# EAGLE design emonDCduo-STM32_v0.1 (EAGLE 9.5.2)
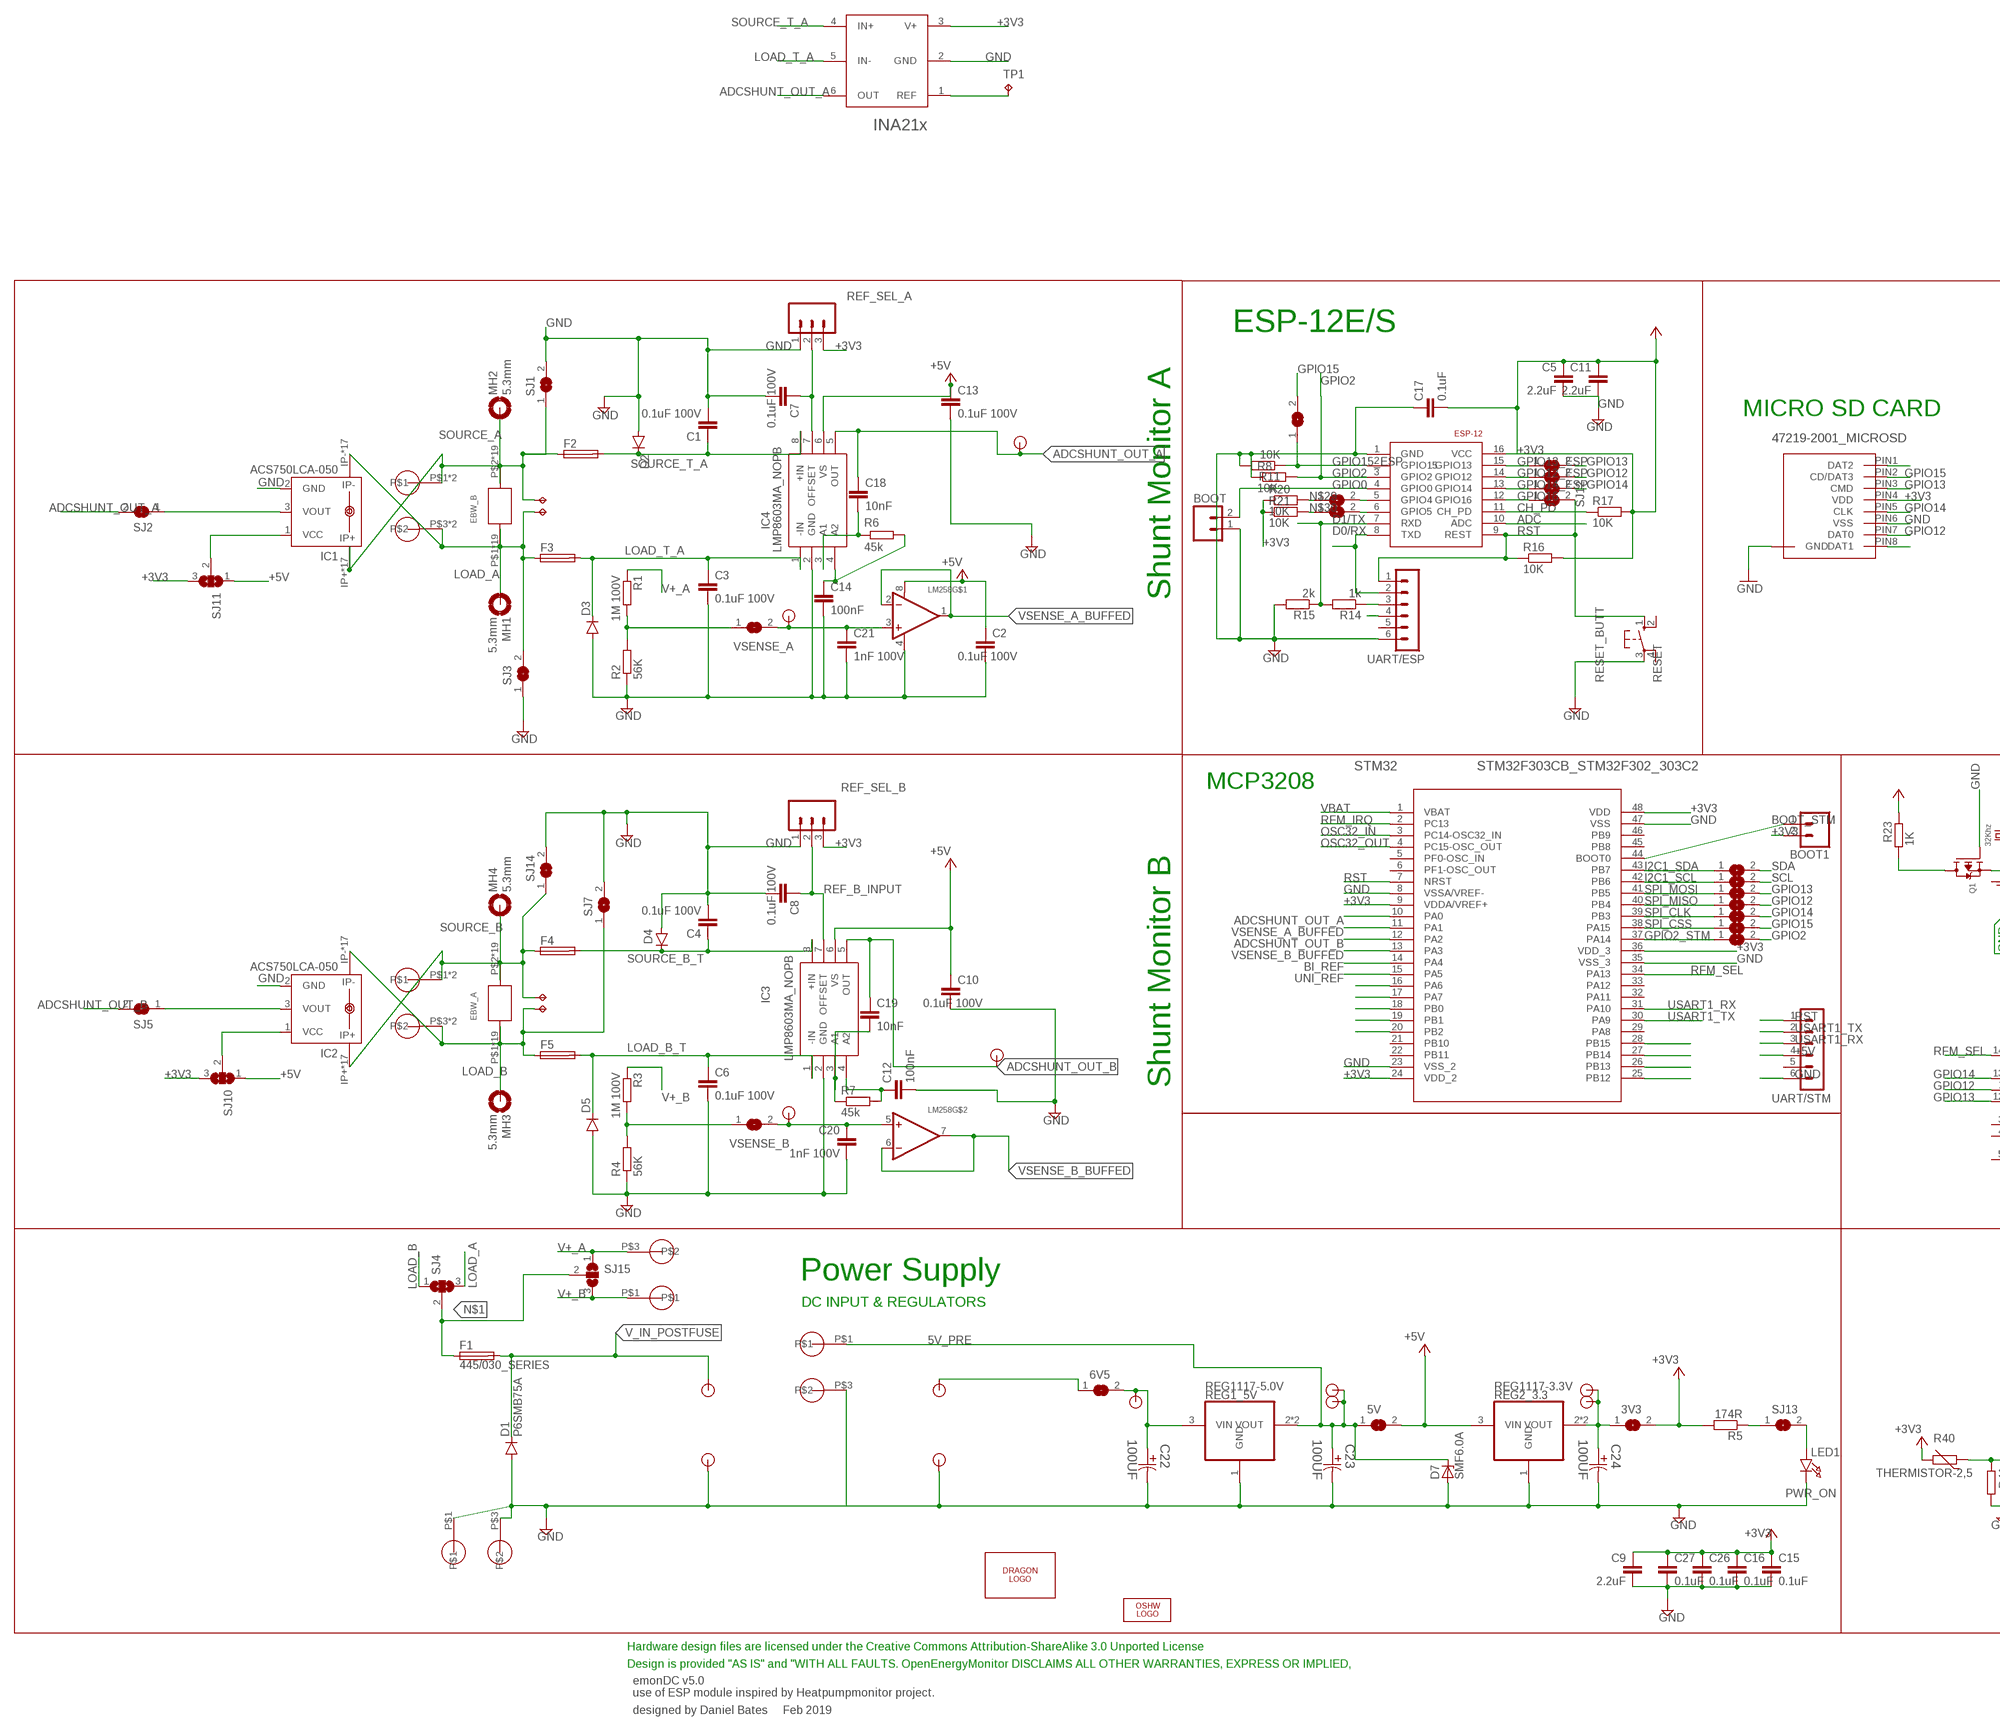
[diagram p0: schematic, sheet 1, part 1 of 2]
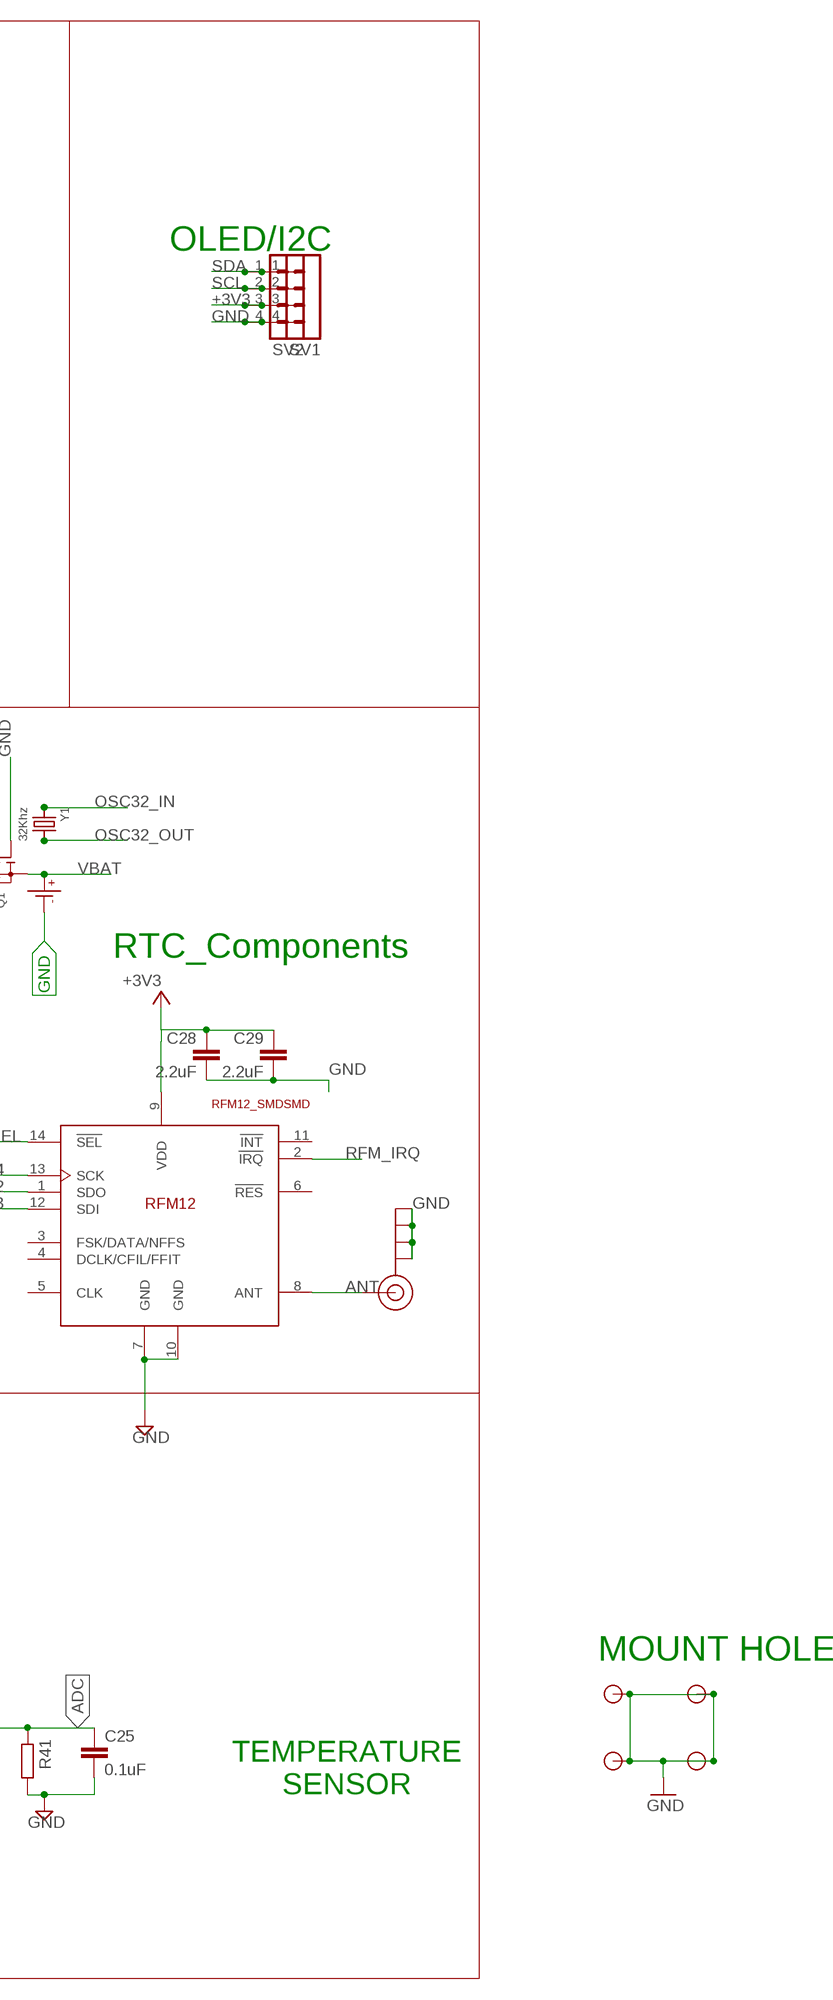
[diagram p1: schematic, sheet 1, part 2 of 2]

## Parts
3V3  SOLDERJUMPERCLOSED  [SOLDERJUMPER_CLOSEDWIRE]
5V  SOLDERJUMPERCLOSED  [SOLDERJUMPER_CLOSEDWIRE]
6V5  SOLDERJUMPERCLOSED  [SOLDERJUMPER_CLOSEDWIRE]
BOOT  M02PTH  [1X02]
BOOT1  M02PTH  [1X02]
C1  0.1uF 100V  C-EUC0603  [C0603]
C2  0.1uF 100V  C-EUC0603  [C0603]
C3  0.1uF 100V  C-EUC0603  [C0603]
C4  0.1uF 100V  C-EUC0603  [C0603]
C5  2.2uF  C-EUC0805  [C0805]
C6  0.1uF 100V  C-EUC0603  [C0603]
C7  0.1uF 100V  C-EUC0603  [C0603]
C8  0.1uF 100V  C-EUC0603  [C0603]
C9  2.2uF  C-EUC0805  [C0805]
C10  0.1uF 100V  C-EUC0603  [C0603]
C11  2.2uF  C-EUC0805  [C0805]
C12  100nF  C-EUC0603  [C0603]
C13  0.1uF 100V  C-EUC0603  [C0603]
C14  100nF  C-EUC0603  [C0603]
C15  0.1uF  C-EUC0603  [C0603]
C16  0.1uF  C-EUC0603  [C0603]
C17  0.1uF  C-EUC0603  [C0603]
C18  10nF  C-EUC0603  [C0603]
C19  10nF  C-EUC0603  [C0603]
C20  1nF 100V  C-EUC0603  [C0603]
C21  1nF 100V  C-EUC0603  [C0603]
C22  100UF  EEE-0JA101WAR-CASE-C  [CAPAE530X610N]
C23  100UF  EEE-0JA101WAR-CASE-C  [CAPAE530X610N]
C24  100UF  EEE-0JA101WAR-CASE-C  [CAPAE530X610N]
C25  0.1uF  C-EUC0603  [C0603]
C26  0.1uF  C-EUC0603  [C0603]
C27  0.1uF  C-EUC0603  [C0603]
C28  2.2uF  C-EUC0805  [C0805]
C29  2.2uF  C-EUC0805  [C0805]
CR1220  CR1220SMD  [CR1220SMD]
D1  P6SMB75A  DIODE-DO214AA  [DO214AA]
D2  P6SMB75A  DIODE-SMB  [SMB]
D3  P6SMB75A  DIODE-SMB  [SMB]
D4  P6SMB75A  DIODE-SMB  [SMB]
D5  P6SMB75A  DIODE-SMB  [SMB]
D7  SMF6.0A  [SOD123F]
EBW_A  EBW_SERIES_15.2MM  [EBW_SERIES_15.2MM]
EBW_B  EBW_SERIES_15.2MM  [EBW_SERIES_15.2MM]
ESP-12  ESP8266_ESP-12  [ESP8266-ESP12]
F1  445/030_SERIES  [445/030_SERIES_LITTELFUSE]
F2  TR5  [TR5]
F3  TR5  [TR5]
F4  TR5  [TR5]
F5  TR5  [TR5]
IC1  ACS750LCA-050  [ACS75050]
IC2  ACS750LCA-050  [ACS75050]
IC3  LMP8603MA_NOPB  [SOIC127P600X175-8N]
IC4  LMP8603MA_NOPB  [SOIC127P600X175-8N]
INA21X_1  INA21X  [SC70]
J$1  SMA_EDGE  [SMA-EDGE]
LED1  PWR_ON  LED1206  [CHIPLED_1206]
LM258  LM358  [SOIC8_150MIL]
LOGO1  OSHW_LOGO_6MILX0200-NT  [OSHW_6X200_NOTEXT]
MH1  5.3mm  MOUNT-PAD-ROUND5.3  [5,3//11-PAD]
MH2  5.3mm  MOUNT-PAD-ROUND5.3  [5,3//11-PAD]
MH3  5.3mm  MOUNT-PAD-ROUND5.3  [5,3//11-PAD]
MH4  5.3mm  MOUNT-PAD-ROUND5.3  [5,3//11-PAD]
MICRO_SD  47219-2001_MICROSD  [47219-2001_MICROSD]
MOUNT_10.16_A  MOLEX_39970-003  [2/10,16]
MOUNT_10.16_B  MOLEX_39970-003  [2/10,16]
Q1  MOSFET-P  [SOT23-R]
R1  1M 100V  R-EU_0207/2V  [0207/2V]
R2  56K  R-EU_0207/2V  [0207/2V]
R3  1M 100V  R-EU_0207/2V  [0207/2V]
R4  56K  R-EU_0207/2V  [0207/2V]
R5  174R  R-EU_R0603  [R0603]
R6  45k  R-EU_R0603  [R0603]
R7  45k  R-EU_R0603  [R0603]
R8  10K  R-EU_R0603  [R0603]
R11  10K  R-EU_R0603  [R0603]
R14  1k  R-EU_R0603  [R0603]
R15  2k  R-EU_R0603  [R0603]
R16  10K  R-EU_R0603  [R0603]
R17  10K  R-EU_R0603  [R0603]
R20  10K  R-EU_R0603  [R0603]
R21  10K  R-EU_R0603  [R0603]
R23  1K  R-EU_R0603  [R0603]
R40  THERMISTOR-2,5  [RS-2,5]
R41  R-EU_0207/2V  [0207/2V]
REF_SEL_A  455-1750-1-ND  CONN_03  [1X03]
REF_SEL_B  455-1750-1-ND  CONN_03  [1X03]
REG1_5V  REG1117-5.0V  REG1117  [SOT223]
REG2_3.3  REG1117-3.3V  REG1117  [SOT223]
RESET  RESET_BUTT  10-XX  [B3F-10XX]
SJ1  SJ  [SJ]
SJ2  SJ  [SJ]
SJ3  SJ  [SJ]
SJ4  SJ2W  [SJ_2]
SJ5  SJ  [SJ]
SJ6  SJTINY  [SJ-SMALL]
SJ7  SJ  [SJ]
SJ8  SOLDERJUMPERCLOSED  [SOLDERJUMPER_CLOSEDWIRE]
SJ9  SOLDERJUMPERCLOSED  [SOLDERJUMPER_CLOSEDWIRE]
SJ10  SJ2W  [SJ_2]
SJ11  SJ2W  [SJ_2]
SJ12  SJTINY  [SJ-SMALL]
SJ13  SOLDERJUMPERCLOSED  [SOLDERJUMPER_CLOSEDWIRE]
SJ14  SJ  [SJ]
SJ15  SJ2W  [SJ_2]
SJ16  SJTINY  [SJ-SMALL]
SJ17  SJTINY  [SJ-SMALL]
SJ18  SJTINY  [SJ-SMALL]
SJ19  SJTINY  [SJ-SMALL]
SJ20  SJTINY  [SJ-SMALL]
SJ21  SJTINY  [SJ-SMALL]
SJ22  SJTINY  [SJ-SMALL]
SJ23  SJTINY  [SJ-SMALL]
SJ24  SJTINY  [SJ-SMALL]
SJ25  SJTINY  [SJ-SMALL]
SJ26  SJTINY  [SJ-SMALL]
SJ27  SJTINY  [SJ-SMALL]
STM32  STM32F303CB_STM32F302_303C2  [STM32F303CB_LQFP48-7X7MM]
SV1  MA04-1  [MA04-1]
SV2  MA04-1  [MA04-1]
TP1  TPPAD1-13  [P1-13]
TP8  TPPAD1-13Y  [P1-13Y]
TP9  TPPAD1-13Y  [P1-13Y]
TP10  TPPAD1-13Y  [P1-13Y]
TP11  TPPAD1-13Y  [P1-13Y]
U$1  TP0.8MM  [TP0.8]
U$2  2212S-02SG-85  TP_2_LONG  [TP0.8_X2]
U$3  2212S-02SG-85  TP_2_LONG  [TP0.8_X2]
U$4  TP0.8MM  [TP0.8]
U$5  TP0.8MM  [TP0.8]
U$6  TP0.8MM  [TP0.8]
U$7  TP0.8MM  [TP0.8]
U$8  TP0.8MM  [TP0.8]
U$9  TP0.8MM  [TP0.8]
U$10  2212S-02SG-85  TP_2_LONG  [TP0.8_X2]
U$11  2212S-02SG-85  TP_2_LONG  [TP0.8_X2]
U$12  5MMBLOCK  [2/5.08]
U$13  5MMBLOCK  [2/5.08]
U$14  RFM12_SMDSMD  [RFM12]
U$18  TP0.8MM  [TP0.8]
U$19  TP0.8MM  [TP0.8]
U$21  5MMBLOCK  [2/5.08]
U$22  TP3.5MM  [TP3.5]
U$23  TP3.5MM  [TP3.5]
U$24  TP3.5MM  [TP3.5]
U$25  TP3.5MM  [TP3.5]
U$26  DRAGON  [DRAGON_LOGO]
UART/ESP  UART/ESP  MA06-1  [MA06-1]
UART/STM  UART/STM  MA06-1  [MA06-1]
Y1  32Khz  CRYSTAL8X3.8SMT  [CRYSTAL_8X3.8]

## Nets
3.3V_PRE [thick_power]: 3V3.1 C24.1 REG2_3.3.2(VOUT) REG2_3.3.4(VOUT) U$8.P$1 U$19.P$1
5V_PRE [thick_power]: 5V.1 C23.1 D7.C REG1_5V.2(VOUT) REG1_5V.4(VOUT) U$7.P$1 U$12.P$1 U$18.P$1
6.5V [thick_power]: 6V5.2 C22.1 REG1_5V.3(VIN) U$9.P$1
+3V3 [thin_power]: 3V3.2 BOOT1.2 C5.1 C9.1 C11.1 C15.1 C16.1 C17.2 C26.1 C27.1 C28.1 C29.1 ESP-12.16(VCC) INA21X_1.3(V+) MICRO_SD.PIN4(VDD) R5.2 R16.2 R17.2 R20.1 R21.1 R23.2 R40.2 REF_SEL_A.3 REF_SEL_B.3 SJ10.3 SJ11.3 STM32.9(VDDA/VREF+) STM32.24(VDD_2) STM32.36(VDD_3) STM32.48(VDD) SV1.3 SV2.3 U$14.9(VDD)
+3V3_BAT [thick_power]: Q1.3(D) R23.1
+5V [thick_power]: 5V.2 C2.1 C10.1 C13.1 IC3.6(VS) IC4.6(VS) LM258.8(V+) REG2_3.3.3(VIN) SJ10.1 SJ11.1 UART/ESP.4 UART/STM.4
ADC: C25.1 ESP-12.10(ADC) R40.1 R41.2
ADCSHUNT_OUT_A: C18.1 IC4.5(OUT) INA21X_1.6(OUT) SJ2.2 STM32.10(PA0) U$6.P$1
ADCSHUNT_OUT_B: C19.1 IC3.5(OUT) SJ5.2 STM32.12(PA2) U$5.P$1
ANT: J$1.SIG(SIGNAL) U$14.8(ANT)
BI_REF: STM32.14(PA4)
BOOT_STM: BOOT1.1 STM32.44(BOOT0)
CH_PD: ESP-12.11(CH_PD) R17.1
D0/RX: ESP-12.8(TXD) UART/ESP.2
D1/TX: ESP-12.7(RXD) R14.2 R15.1
GND: BOOT.1 C1.2 C2.2 C3.2 C4.2 C5.2 C6.2 C7.2 C8.2 C9.2 C10.2 C11.2 C12.2 C13.2 C14.2 C15.2 C16.2 C17.1 C20.2 C21.2 C22.2 C23.2 C24.2 C25.2 C26.2 C27.2 C28.2 C29.2 CR1220.P-(P$-) D1.A D2.A D3.A D4.A D5.A D7.A ESP-12.1(GND) IC1.2(GND) IC2.2(GND) IC3.2(GND) IC4.2(GND) INA21X_1.2(GND) J$1.GND@0(GND) J$1.GND@1(GND) J$1.GND@2(GND) J$1.GND@3(GND) LED1.C LM258.4(V-) MICRO_SD.P$1(GND) MICRO_SD.P$2(GND) MICRO_SD.P$3(GND) MICRO_SD.P$4(GND) MICRO_SD.PIN6(VSS) Q1.1(G) R2.1 R4.1 R8.1 R11.2 R15.2 R41.1 REF_SEL_A.1 REF_SEL_B.1 REG1_5V.1(GND) REG2_3.3.1(GND) RESET.3(P) SJ1.2 SJ3.1 SJ7.2 SJ14.2 STM32.8(VSSA/VREF-) STM32.23(VSS_2) STM32.35(VSS_3) STM32.47(VSS) SV1.4 SV2.4 U$3.P$1 U$3.P$2 U$11.P$1 U$11.P$2 U$12.P$3 U$13.P$1 U$13.P$3 U$14.7(GND) U$14.10(GND) U$22.P$1 U$23.P$1 U$24.P$1 U$25.P$1 UART/ESP.6 UART/STM.6
GPIO0: BOOT.2 ESP-12.4(GPIO0)
GPIO2: ESP-12.3(GPIO2) R8.2 SJ21.2
GPIO2_STM: SJ21.1 STM32.37(PA14)
GPIO12: MICRO_SD.PIN7(DAT0) SJ17.2 SJ26.2 U$14.1(SDO)
GPIO12_ESP: ESP-12.14(GPIO12) SJ26.1
GPIO13: MICRO_SD.PIN3(CMD) SJ18.2 SJ25.2 U$14.12(SDI)
GPIO13_ESP: ESP-12.15(GPIO13) SJ25.1
GPIO14: MICRO_SD.PIN5(CLK) SJ16.2 SJ27.2 U$14.13(SCK)
GPIO14_ESP: ESP-12.13(GPIO14) SJ27.1
GPIO15: MICRO_SD.PIN2(CD/DAT3) SJ6.2 SJ22.2
GPIO15_ESP: ESP-12.2(GPIO15) R11.1 SJ22.1
GPIO16: ESP-12.12(GPIO16) SJ12.1
I2C1_SCL: SJ19.1 STM32.42(PB6)
I2C1_SDA: SJ20.1 STM32.43(PB7)
LOAD_A [HV]: EBW_B.P$1 EBW_B.P$3 EBW_B.P$4 EBW_B.P$5 EBW_B.P$6 EBW_B.P$7 EBW_B.P$8 EBW_B.P$9 EBW_B.P$10 EBW_B.P$11 EBW_B.P$12 EBW_B.P$13 EBW_B.P$14 EBW_B.P$15 EBW_B.P$16 EBW_B.P$17 EBW_B.P$33 EBW_B.P$34 EBW_B.P$35 F3.1 IC1.IP- IC1.IP-@2(IP-) IC1.IP-@3(IP-) IC1.IP-@4(IP-) IC1.IP-@5(IP-) IC1.IP-@6(IP-) IC1.IP-@7(IP-) IC1.IP-@8(IP-) IC1.IP-@9(IP-) IC1.IP-@10(IP-) IC1.IP-@11(IP-) IC1.IP-@12(IP-) IC1.IP-@13(IP-) IC1.IP-@14(IP-) IC1.IP-@15(IP-) IC1.IP-@16(IP-) IC1.IP-@17(IP-) MH1.B5,5(MOUNT) MOUNT_10.16_A.P$3 MOUNT_10.16_A.P$4 SJ3.2 SJ4.3 TP10.TP
LOAD_B [HV]: EBW_A.P$1 EBW_A.P$3 EBW_A.P$4 EBW_A.P$5 EBW_A.P$6 EBW_A.P$7 EBW_A.P$8 EBW_A.P$9 EBW_A.P$10 EBW_A.P$11 EBW_A.P$12 EBW_A.P$13 EBW_A.P$14 EBW_A.P$15 EBW_A.P$16 EBW_A.P$17 EBW_A.P$33 EBW_A.P$34 EBW_A.P$35 F5.1 IC2.IP- IC2.IP-@2(IP-) IC2.IP-@3(IP-) IC2.IP-@4(IP-) IC2.IP-@5(IP-) IC2.IP-@6(IP-) IC2.IP-@7(IP-) IC2.IP-@8(IP-) IC2.IP-@9(IP-) IC2.IP-@10(IP-) IC2.IP-@11(IP-) IC2.IP-@12(IP-) IC2.IP-@13(IP-) IC2.IP-@14(IP-) IC2.IP-@15(IP-) IC2.IP-@16(IP-) IC2.IP-@17(IP-) MH3.B5,5(MOUNT) MOUNT_10.16_B.P$3 MOUNT_10.16_B.P$4 SJ4.1 SJ7.1 TP8.TP
LOAD_B_T [thin_power]: C6.1 D5.C F5.2 IC3.1(-IN)
LOAD_T_A [thin_power]: C3.1 D3.C F3.2 IC4.1(-IN) INA21X_1.5(IN-)
N$1: F1.P$1 F1.P$2 SJ4.2 SJ15.2
N$3: C14.1 IC4.4(A2) R6.2
N$4: C18.2 IC4.3(A1) R6.1
N$5: R5.1 SJ13.1
N$6: LED1.A SJ13.2
N$7: MICRO_SD.PIN1(DAT2)
N$9: STM32.18(PB0)
N$10: STM32.19(PB1)
N$11: STM32.20(PB2)
N$15: STM32.25(PB12)
N$17: STM32.26(PB13)
N$20: STM32.27(PB14)
N$22: STM32.28(PB15)
N$23: STM32.17(PA7)
N$24: STM32.16(PA6)
N$25: C19.2 IC3.3(A1) R7.1
N$27: C12.1 IC3.4(A2) R7.2
N$29: R20.2 SJ23.1
N$30: R21.2 SJ24.1
N$32: MICRO_SD.PIN8(DAT1)
N$36: R14.1 UART/ESP.3
N$37: INA21X_1.1(REF) TP1.TP
OSC32_IN: STM32.3(PC14-OSC32_IN) Y1.P$1
OSC32_OUT: STM32.4(PC15-OSC_OUT) Y1.P$4
REF_A_INPUT: C7.1 IC4.7(OFFSET) REF_SEL_A.2
REF_B_INPUT: C8.1 IC3.7(OFFSET) REF_SEL_B.2
RFM_IRQ: STM32.2(PC13) U$14.2(!IRQ)
RFM_SEL: STM32.34(PA13) U$14.14(!SEL)
RST: ESP-12.9(REST) R16.1 RESET.1(S) SJ12.2 STM32.7(NRST) UART/ESP.1 UART/STM.1
SCL: ESP-12.6(GPIO5) SJ19.2 SJ24.2 SV1.2 SV2.2
SDA: ESP-12.5(GPIO4) SJ20.2 SJ23.2 SV1.1 SV2.1
SOURCE_A [HV]: EBW_B.P$2 EBW_B.P$18 EBW_B.P$19 EBW_B.P$20 EBW_B.P$21 EBW_B.P$22 EBW_B.P$23 EBW_B.P$24 EBW_B.P$25 EBW_B.P$26 EBW_B.P$27 EBW_B.P$28 EBW_B.P$29 EBW_B.P$30 EBW_B.P$31 EBW_B.P$32 EBW_B.P$36 EBW_B.P$37 EBW_B.P$38 F2.1 IC1.IP+ IC1.IP+@2(IP+) IC1.IP+@3(IP+) IC1.IP+@4(IP+) IC1.IP+@5(IP+) IC1.IP+@6(IP+) IC1.IP+@7(IP+) IC1.IP+@8(IP+) IC1.IP+@9(IP+) IC1.IP+@10(IP+) IC1.IP+@11(IP+) IC1.IP+@12(IP+) IC1.IP+@13(IP+) IC1.IP+@14(IP+) IC1.IP+@15(IP+) IC1.IP+@16(IP+) IC1.IP+@17(IP+) MH2.B5,5(MOUNT) MOUNT_10.16_A.P$1 MOUNT_10.16_A.P$2 SJ1.1 TP11.TP
SOURCE_B [HV]: EBW_A.P$2 EBW_A.P$18 EBW_A.P$19 EBW_A.P$20 EBW_A.P$21 EBW_A.P$22 EBW_A.P$23 EBW_A.P$24 EBW_A.P$25 EBW_A.P$26 EBW_A.P$27 EBW_A.P$28 EBW_A.P$29 EBW_A.P$30 EBW_A.P$31 EBW_A.P$32 EBW_A.P$36 EBW_A.P$37 EBW_A.P$38 F4.1 IC2.IP+ IC2.IP+@2(IP+) IC2.IP+@3(IP+) IC2.IP+@4(IP+) IC2.IP+@5(IP+) IC2.IP+@6(IP+) IC2.IP+@7(IP+) IC2.IP+@8(IP+) IC2.IP+@9(IP+) IC2.IP+@10(IP+) IC2.IP+@11(IP+) IC2.IP+@12(IP+) IC2.IP+@13(IP+) IC2.IP+@14(IP+) IC2.IP+@15(IP+) IC2.IP+@16(IP+) IC2.IP+@17(IP+) MH4.B5,5(MOUNT) MOUNT_10.16_B.P$1 MOUNT_10.16_B.P$2 SJ14.1 TP9.TP
SOURCE_B_T [thin_power]: C4.1 D4.C F4.2 IC3.8(+IN)
SOURCE_T_A [thin_power]: C1.1 D2.C F2.2 IC4.8(+IN) INA21X_1.4(IN+)
SPI_CLK: SJ16.1 STM32.39(PB3)
SPI_CSS: SJ6.1 STM32.38(PA15)
SPI_MISO: SJ17.1 STM32.40(PB4)
SPI_MOSI: SJ18.1 STM32.41(PB5)
UNI_REF: STM32.15(PA5)
USART1_RX: STM32.31(PA10) UART/STM.3
USART1_TX: STM32.30(PA9) UART/STM.2
V+_A [HV]: R1.1 SJ15.1 U$21.P$3
V+_B [HV]: R3.1 SJ15.3 U$21.P$1
V_IN_POSTFUSE [HV]: D1.C F1.P$3 F1.P$4 U$2.P$1 U$2.P$2
VBAT: CR1220.P+(P$+) Q1.2(S) STM32.1(VBAT)
VCC_ACS_A: IC1.1(VCC) SJ11.2
VCC_ACS_B: IC2.1(VCC) SJ10.2
VOUT_ACS_A: IC1.3(VOUT) SJ2.1
VOUT_ACS_B: IC2.3(VOUT) SJ5.1
VOUT_POST_SWITCHING: 6V5.1 U$10.P$1 U$10.P$2
VSENSE_A: R1.2 R2.2 SJ8.1
VSENSE_A_BUFFED: LM258.1(OUT) LM258.2(-IN) STM32.11(PA1)
VSENSE_A_TP: C21.1 LM258.3(+IN) SJ8.2 U$1.P$1
VSENSE_B: R3.2 R4.2 SJ9.1
VSENSE_B_BUFFED: LM258.6(-IN) LM258.7(OUT) STM32.13(PA3)
VSENSE_B_TP: C20.1 LM258.5(+IN) SJ9.2 U$4.P$1
Unconnected: RESET.2(S1) RESET.4(P1) STM32.5(PF0-OSC_IN) STM32.6(PF1-OSC_OUT) STM32.21(PB10) STM32.22(PB11) STM32.29(PA8) STM32.32(PA11) STM32.33(PA12) STM32.45(PB8) STM32.46(PB9) U$14.3(FSK/DATA/NFFS) U$14.4(DCLK/CFIL/FFIT) U$14.5(CLK) U$14.6(!RES) U$14.11(!INT) UART/ESP.5 UART/STM.5

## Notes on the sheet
- ESP-12E/S
- MICRO SD CARD
- OLED/I2C
- Shunt Monitor A
- MCP3208
- RTC_Components
- Shunt Monitor B
- Power Supply
- DC INPUT & REGULATORS
- MOUNT HOLES
- TEMPERATURE
  SENSOR
- Hardware design files are licensed under the Creative Commons Attribution-ShareAlike 3.0 Unported License
- Design is provided "AS IS" and "WITH ALL FAULTS. OpenEnergyMonitor DISCLAIMS ALL OTHER WARRANTIES, EXPRESS OR IMPLIED,
- emonDC v5.0
  use of ESP module inspired by Heatpumpmonitor project.
- designed by Daniel Bates     Feb 2019

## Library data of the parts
3V3 5V 6V5 SJ8 SJ9 SJ13 = microbuilder:SOLDERJUMPER: SMD Solder JUMPER
BOOT BOOT1 = SparkFun:M02: Header 2
C1-C4 C6-C8 C10 C13 C14 C18-C21 = rcl:C-EU: CAPACITOR, European symbol; MPN: C1608X7S2A104K080AB; SPICEPREFIX: C
C5 C9 C11 C12 C15-C17 C25-C29 = rcl:C-EU: CAPACITOR, European symbol; SPICEPREFIX: C
C22-C24 = Panasonic-EEE0_EEE1_EEE2_EEEFC:EEE-: Aluminum Electrolytic Capacitors,Surface Mount Type; MPN: EEE-0JA101WAR; OC_FARNELL: 2284723; OC_NEWARK: 53W3731; PACKAGE: CASE-C; SUPPLIER: PANASONIC; TOLERANCE: 20%; VOLTAGERATING: 6.3V
CR1220 = IotaWatt_parts:CR1220SMD: CR1220 Battery SMD; MPN: Harwin S8411-45R
D1-D5 = diode:DIODE-: DIODE
D7 = smf_10:SMF*A: SMF Series TVS Diodes; MF: Littelfuse; MPN: SMF6.0A; OC_FARNELL: unknown; OC_NEWARK: unknown
EBW_A EBW_B = EBW series SHUNT:EBW_SERIES_15.2MM
ESP-12 = ESP8266-ESP12:ESP8266_ESP-12
F1 = LITTELFUSE 455:030 SERIES:445/030_SERIES: MPN 04450001N
F2-F5 = fuse_db:TR5: FUSE; MF: LITTELFUSE; MPN: 56000001009; OC_FARNELL: 1185363; OC_NEWARK: unknown
IC1 IC2 = allegro:ACS750*CA-050: Current Sensor display layer 49 Reference in BRD and place VIAs on circles Source: www.allegromicro.com/datafile/0750-050.pdf; MF: ALLEGRO MICROSYSTEMS, INC.; MPN: ACS750LCA-050; OC_FARNELL: 1457176; OC_NEWARK: 61H4464
IC3 IC4 = LMP8603MA_NOPB:LMP8603MA_NOPB: 60-V, Bi-Directional, Low- or High-Side, Voltage Output Current Sensing Amplifier Source: Datasheet; DESCRIPTION: 60-V, Bi-Directional, Low- or High-Side, Voltage Output Current Sensing Amplifier; HEIGHT: 1.75mm; MANUFACTURER_NAME: Texas Instruments; MANUFACTURER_PART_NUMBER: LMP8603MA/NOPB; RS_PART_NUMBER: 7616334P; RS_PRICE-STOCK: http://uk.rs-online.com/web/p/products/7616334P
INA21X_1 = ina21x:INA21X: Texas Instruments INA21x
J$1 = SparkFun-Connectors:SMA_EDGE: SMA Antenna Connector End launch SMA connector. The paste layer has been removed so that the connector can be hand soldered onto the board after reflow.
LED1 = microbuilder:LED: LED
LM258 = microbuilder:LM358: LM358 Dual Operational Amplifier Digikey: LM358AMXFSCT-ND
LOGO1 = ohw-logo:OSHW_LOGO_6MIL; OC_FARNELL: unknown
MH1-MH4 = holes-db:MOUNT-PAD-ROUND: MOUNTING PAD, round
MICRO_SD = MOLEX 47219-2001:47219-2001_MICROSD
MOUNT_10.16_A MOUNT_10.16_B = 10.16mm terminal block:MOLEX_39970-003
Q1 = microbuilder:MOSFET-P: P-Channel Mosfet LEGEND VDS: Voltage Drain-Source ID: Drain Current RDS(ON): Drain-Source On-State Resistance VGS(TH): Gate-Source Threshold Voltage CISS: Drain-Source Input Capacitance SOT-23 Name VDS ID RDS(ON) VGS(TH) CISS Order Number IRLML5103 30V 760mA 600 mOhm -- 75pF @ 25V Digikey: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
R1 R3 = rcl7:R-EU_: RESISTOR, European symbol; MPN: MCMF006FF1004A50
R2 R4 = rcl7:R-EU_: RESISTOR, European symbol; MPN: MCMF006FF7502A50
R5 = rcl:R-EU_: RESISTOR, European symbol; SPICEPREFIX: R
R6-R8 R11 R14-R17 R20 R21 = rcl:R-EU_: RESISTOR, European symbol
R23 = rcl@1:R-EU_: RESISTOR, European symbol
R40 = varistor:THERMISTOR: THERMISTOR
R41 = rcl7:R-EU_: RESISTOR, European symbol
REF_SEL_A REF_SEL_B = SparkFun-Connectors:CONN_03: Multi connection point. Often used as Generic Header-pin footprint for 0.1 inch spaced/style header connections On any of the 0.1 inch spaced packages, you can populate with these: Break Away Headers - Straight (PRT-00116) Break Away Male Headers - Right Angle (PRT-00553) Female Headers (PRT-00115)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; MF: MULTICOMP; MPN: 2212S-02SG-85; OC_FARNELL: 1593458; PROD_ID: XXX-00000
REG1_5V = burr-brown-db:REG1117: 800mA and 1A Low Dropout (LDO) Positive Regulator 1.8V, 2.5V, 2.85V, 3.3V, 5V, and Adj; MF: TEXAS INSTRUMENTS; MPN: REG1117-5.0; OC_FARNELL: 1097566; OC_NEWARK: 14P6981
REG2_3.3 = burr-brown-db:REG1117: 800mA and 1A Low Dropout (LDO) Positive Regulator 1.8V, 2.5V, 2.85V, 3.3V, 5V, and Adj; MF: TEXAS INSTRUMENTS; MPN: REG1117-3.3; OC_FARNELL: 1097566; OC_NEWARK: 14P6981
RESET = switch-omron:10-XX: OMRON SWITCH; MPN: FSM4JH; OC_FARNELL: 155598
SJ1-SJ3 SJ5 SJ7 SJ14 = jumper:SJ: SMD solder JUMPER
SJ4 SJ10 SJ11 SJ15 = jumper:SJ2W: SMD solder JUMPER
SJ6 SJ12 SJ16-SJ27 = jumper-con_db:SJ: SMD solder JUMPER
STM32 = stm32hw05:STM32F303CB_STM32F302_303C2; MANUFACTURER_PART_NUMBER: stm32f302_303c2; VENDOR: STMicroelectronics
SV1 SV2 = con-lstb-db:MA04-1: PIN HEADER; MF: MULTICOMP; MPN: 2212S-04SG-85; OC_FARNELL: 1593460; OC_NEWARK: unknown
TP1 TP8-TP11 = testpad:TP: Test pad
U$1 U$4-U$9 U$18 U$19 U$22-U$25 = testpad_db:TP
U$2 U$3 U$10 U$11 = testpad_db:TP_2_LONG; MPN: 2212S-02SG-85
U$12 U$13 U$21 = 5mm terminal block:5MMBLOCK; MF: LUMBERG; MPN: KRM_02; OC_FARNELL: 1177875
U$14 = rfm12b _ rfm69cw:RFM12_SMD: RFM12 is a low costing ISM band transceiver module implemented with unique PLL. It works signal ranges from 315/433/868/915MHZ bands, comply with FCC, ETSI regulation. The SPI interface is used to communicate with microcontroller for parameter setting.
U$26 = DRAGON_LOGO:DRAGON
UART/ESP UART/STM = JeeLabs:MA06-1: PIN HEADER
Y1 = microbuilder:CRYSTAL: Crystals

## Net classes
0 default: width 0.203 mm, drill 0.5 mm, clearance 0.178 mm
1 power: width 0.254 mm, drill 0.5 mm, clearance 0.203 mm
2 thin_power: width 0.254 mm, drill 0.5 mm, clearance 0.203 mm
3 thick_power: width 0.406 mm, drill 0.5 mm, clearance 0.203 mm
4 HV: width 0.406 mm, drill 0.5 mm, clearance 0.762 mm

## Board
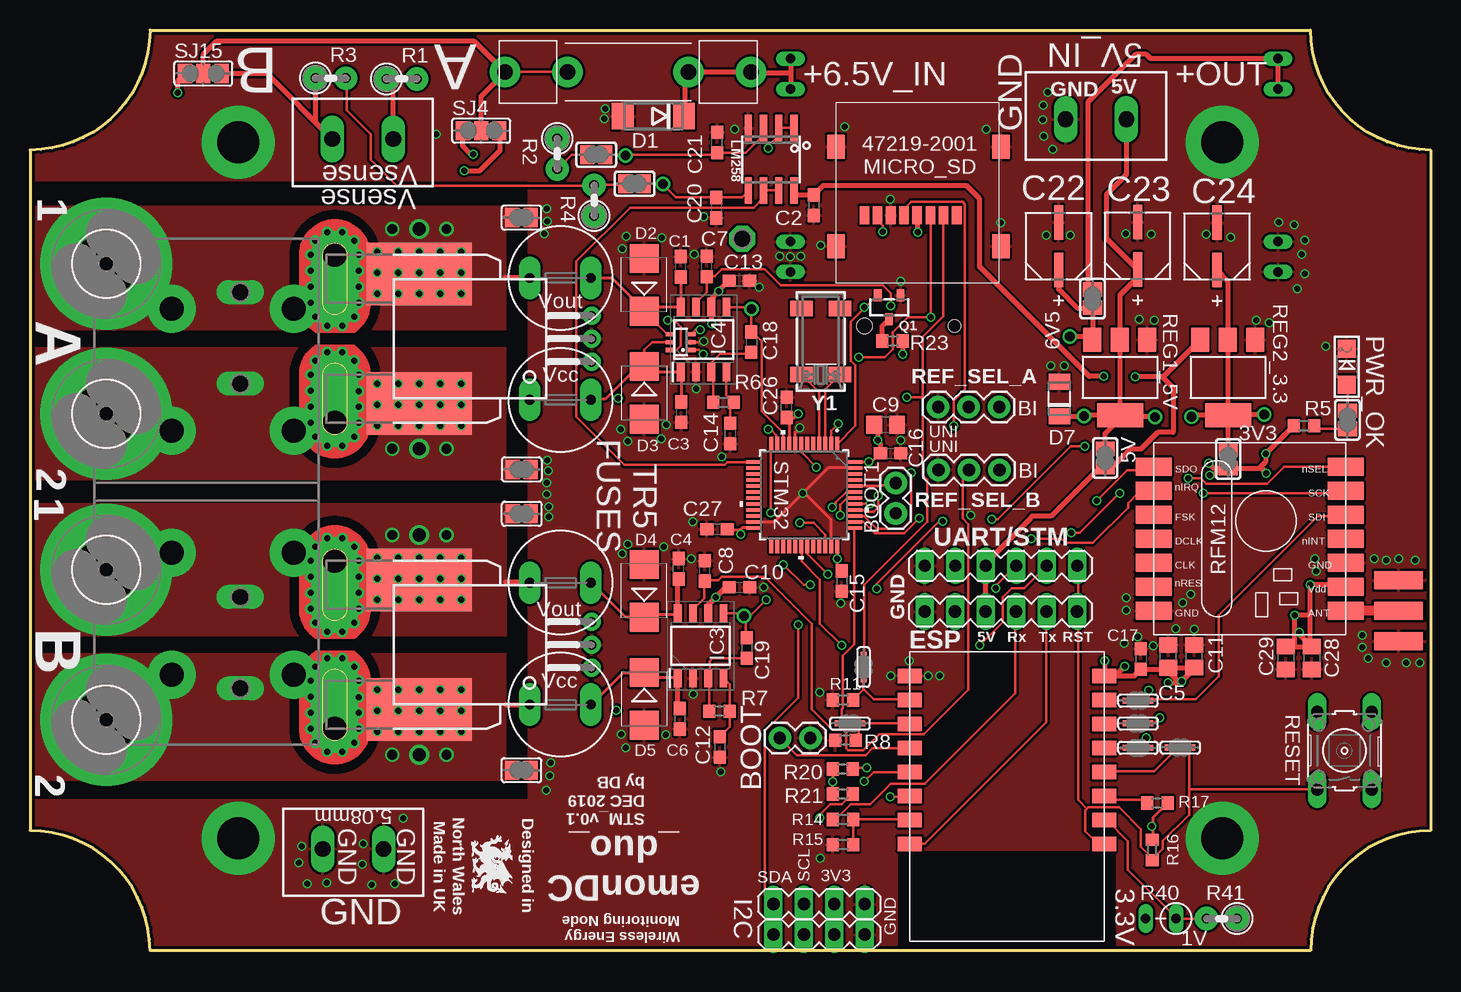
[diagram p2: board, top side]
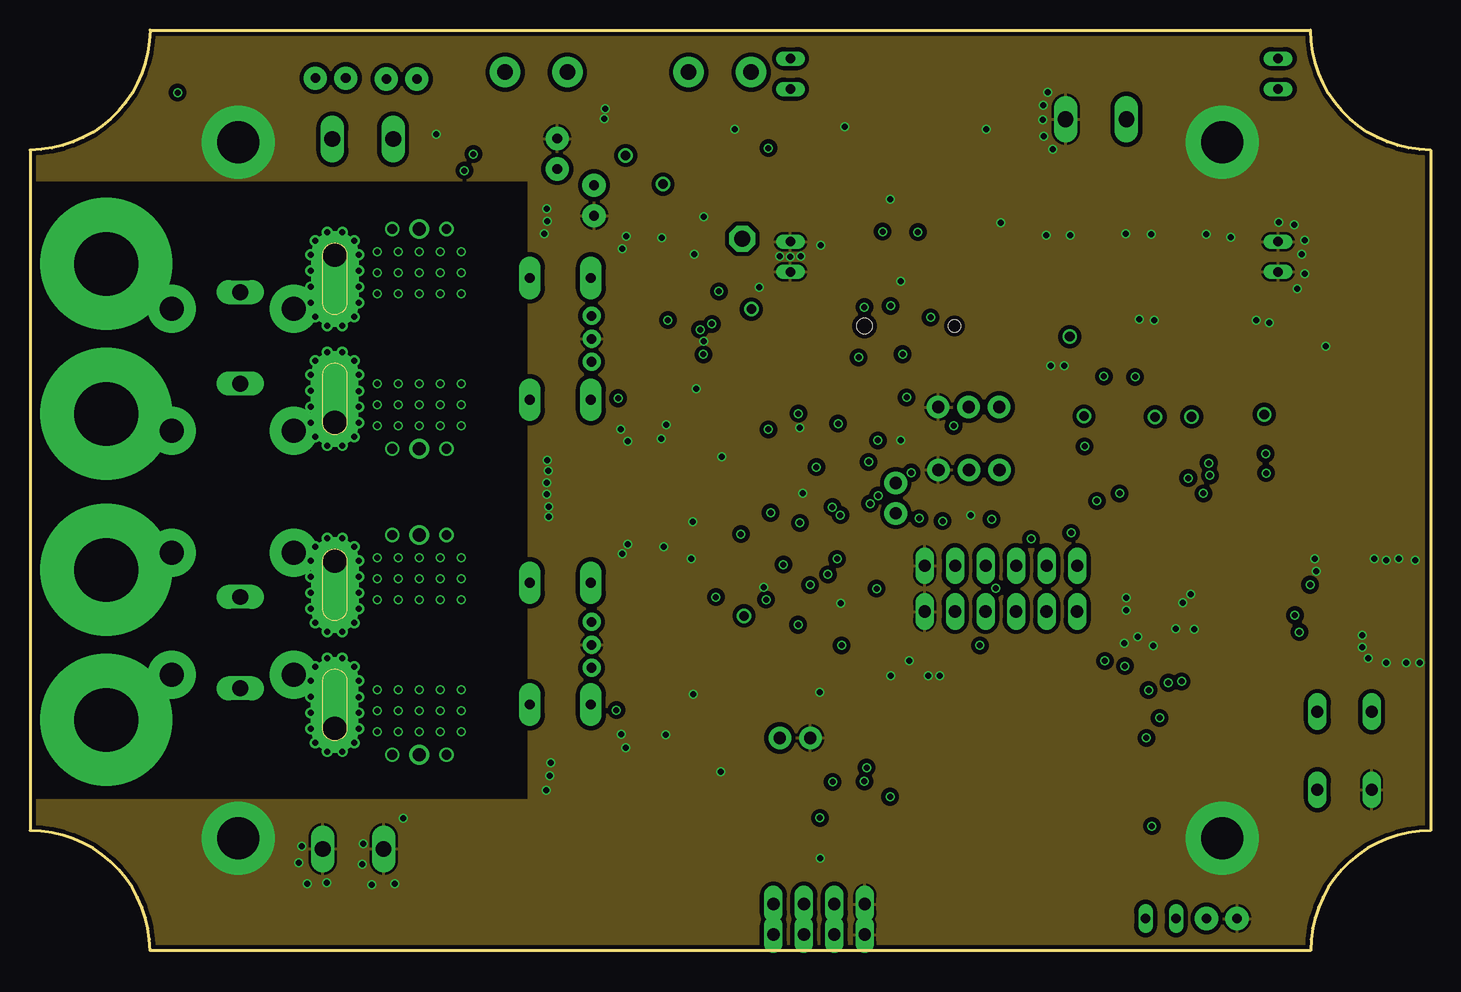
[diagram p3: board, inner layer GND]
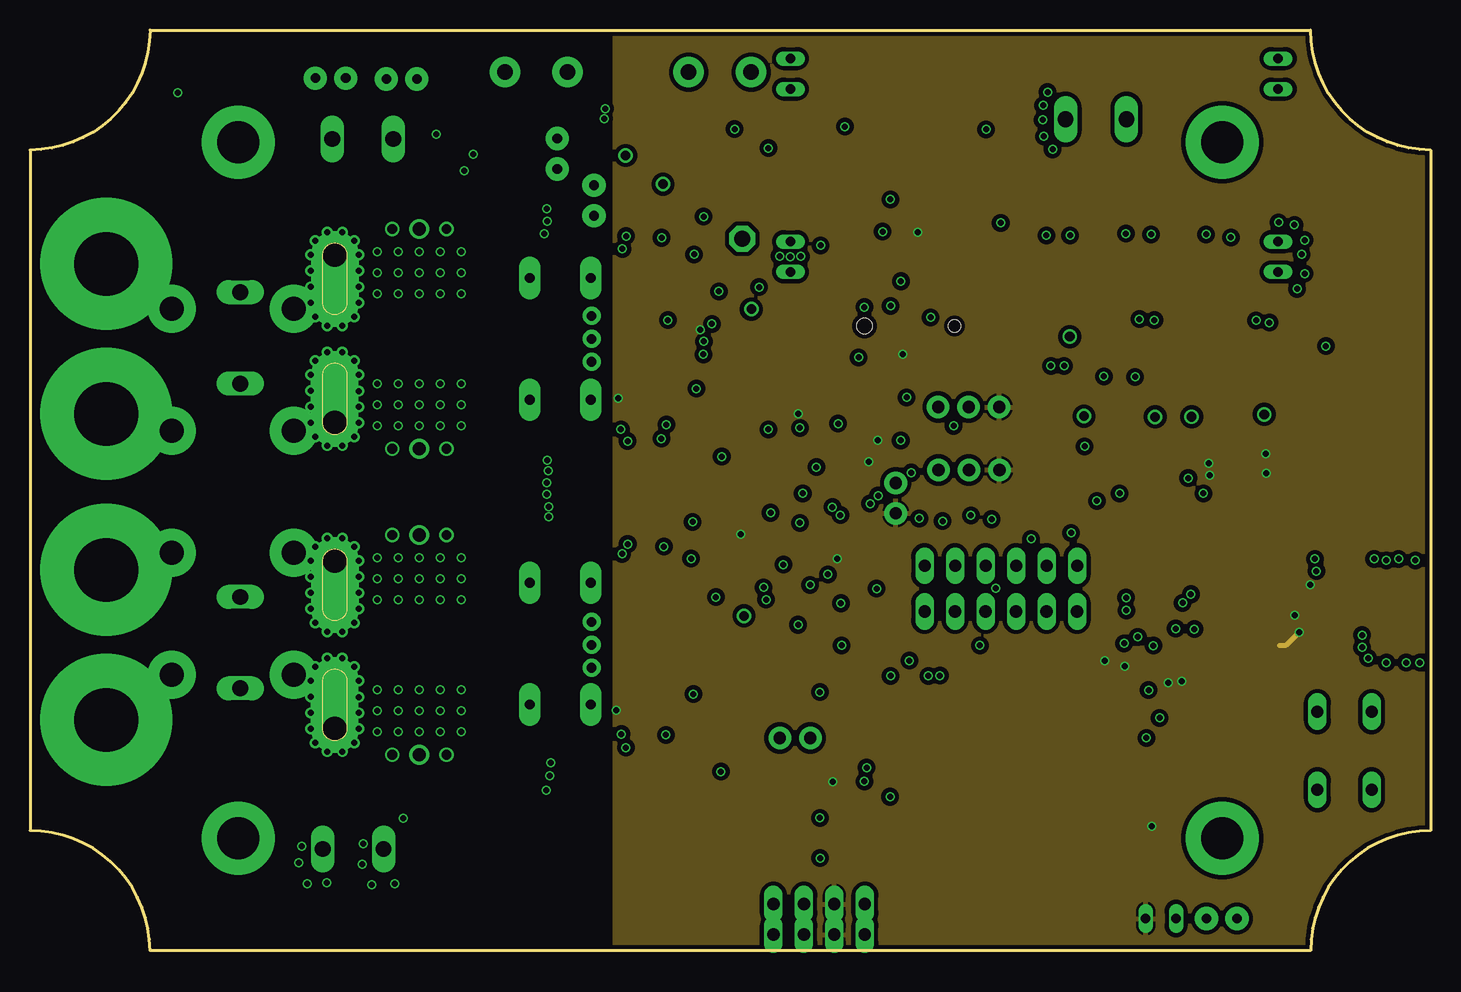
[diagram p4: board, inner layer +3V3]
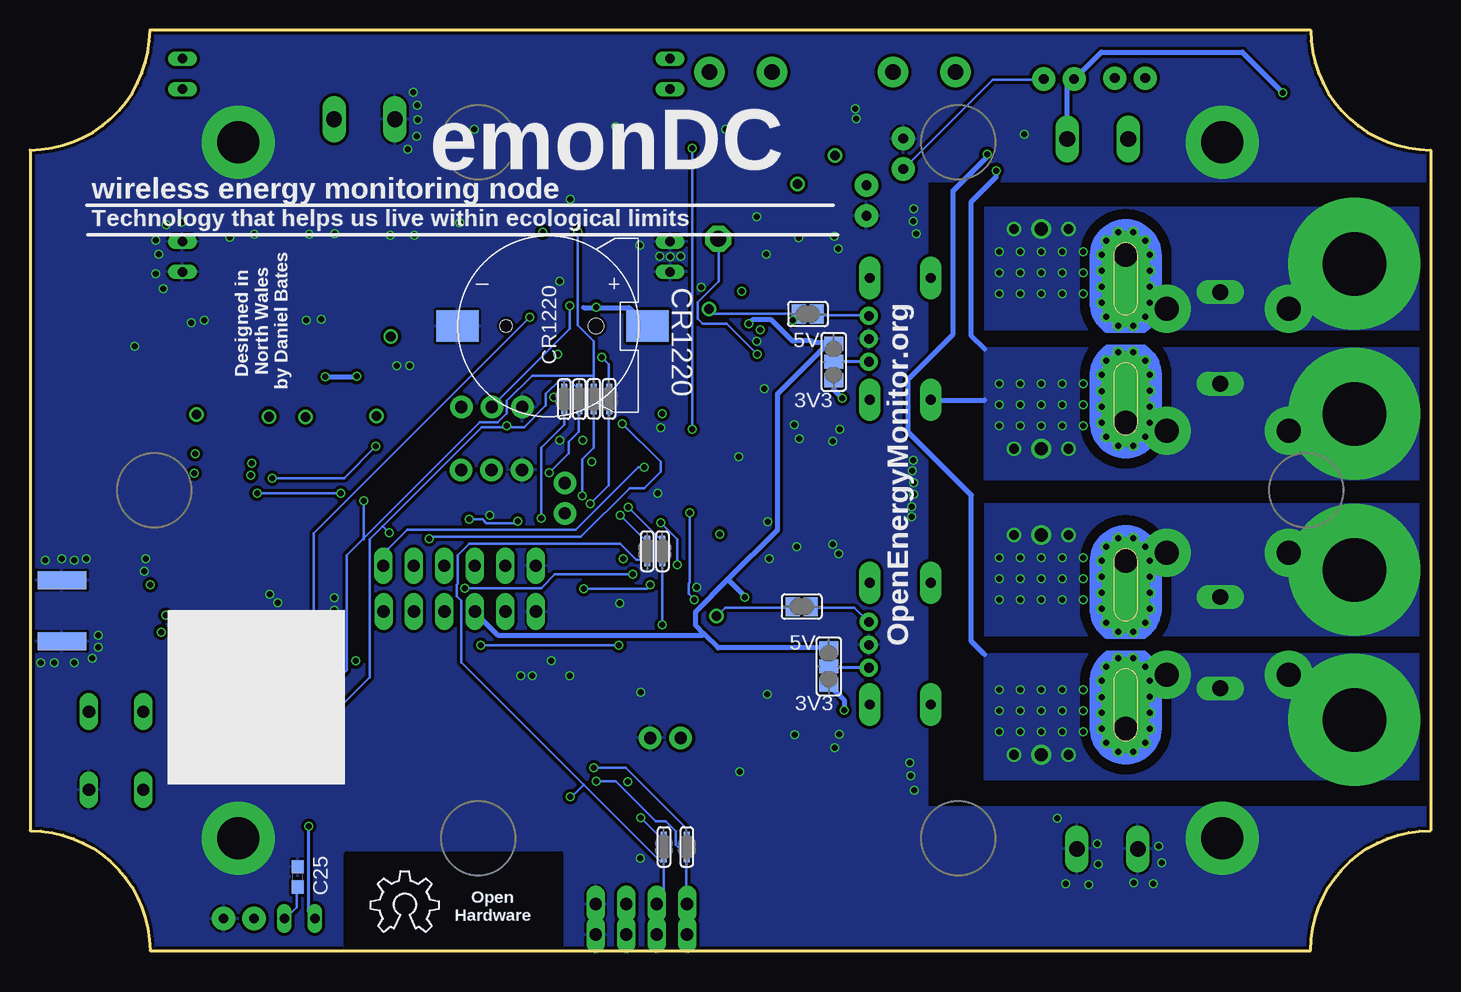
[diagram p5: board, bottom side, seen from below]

Size 116.71 x 76.71 mm. Coordinates in mm from the lower left corner, seen from the top.
Outline: 0,66.71 0,10 arc-90 10,0 106.71,0 arc-90 116.71,10 116.71,66.71 arc-90 106.71,76.71 10,76.71 arc-90 0,66.71
Copper layers (1+2*15+16): Top 0.035mm / dielectric 0.2mm / GND 0.0175mm / dielectric 1.1mm / +3V3 0.0175mm / dielectric 0.2mm / Bottom 0.035mm
Design rules "jlcpcb *": minimum track width 6mil, minimum drill 0.35mm, track to track 7mil, track to pad 7mil, pad to pad 7mil, via to via 0.1mm, smd to smd 2mil, copper to edge 10mil, drill to drill 10mil, minimum pad ring 3mil, minimum via ring 3mil, stop-mask expansion 2mil, vias tented up to drill 25mil, thermal gap 8mil
tRestrict: area 72.5,0.5 to 90.3,8.1
bRestrict: area 72.5,0.4 to 90.3,8

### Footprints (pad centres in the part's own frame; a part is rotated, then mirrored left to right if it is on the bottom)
SOLDERJUMPER_CLOSEDWIRE = smd 1.168 x 1.6: 1 -0.762,0; 2 0.762,0 | smd 0.635 x 0.203: WIRE 0,0
1X02 = drill 1.016 pad 1.88: 1 0,0; 2 2.54,0
C0603 = smd 1.1 x 1: 1 -0.85,0; 2 0.85,0
C0805 = smd 1.3 x 1.5: 1 -0.95,0; 2 0.95,0
CAPAE530X610N = smd 2.87 x 0.762: 1 -1.981,0; 2 1.981,0
CR1220SMD = smd 3.54 x 2.6: P+ 8.3,0; P- -7.55,0 | hole 1: -3.5,0 | hole 1.3: 4,0
DO214AA = smd 1.8 x 2.2: A 2.55,0; C -2.55,0
SMB = smd 2.4 x 2.4: A 2.2,0; C -2.2,0
SOD123F = smd 1.34 x 1.8: A 1.43,0; C -1.43,0
EBW_SERIES_15.2MM = smd 5.2 x 8.75: P$1 -5.4,0; P$2 5.4,0 | drill 0.5: P$3 -3.75,3.5; P$4 -3.75,1.75; P$5 -3.75,0; P$6 -3.75,-1.75; P$7 -3.75,-3.5; P$8 -5.5,3.5; P$9 -5.5,1.75; P$10 -5.5,0; P$11 -5.5,-1.75; P$12 -5.5,-3.5; P$13 -7.25,3.5; P$14 -7.25,1.75; P$15 -7.25,0; P$16 -7.25,-1.75; P$17 -7.25,-3.5; P$18 7.25,1.75; P$19 7.25,3.5; P$20 7.25,0; P$21 7.25,-1.75; P$22 7.25,-3.5; P$23 5.5,3.5; P$24 5.5,1.75; P$25 5.5,0; P$26 5.5,-1.75; P$27 5.5,-3.5; P$28 3.75,3.5; P$29 3.75,1.75; P$30 3.75,0; P$31 3.75,-1.75; P$32 3.75,-3.5 | drill 0.8: P$33 -9.155,2.258; P$35 -9.155,-2.258; P$36 9.155,2.258; P$38 9.155,-2.258 | drill 1.1: P$34 -9.155,0; P$37 9.155,0
ESP8266-ESP12 = smd 2 x 1.2: 1 16.2,2; 2 16.2,4; 3 16.2,6; 4 16.2,8; 5 16.2,10; 6 16.2,12; 7 16.2,14; 8 16.2,16; 9 0,16; 10 0,14; 11 0,12; 12 0,10; 13 0,8; 14 0,6; 15 0,4; 16 0,2
445/030_SERIES_LITTELFUSE = drill 1.3 pad 2.54: P$1 -10.25,0; P$2 -5.05,0; P$3 10.25,0; P$4 5.05,0
TR5 = drill 0.813 pad 1.778 long: 1 -2.54,0; 2 2.54,0
ACS75050 = drill 0.8 pad 1.5: 1 -1.91,-21.4; 2 0,-21.4; 3 1.91,-21.4 | drill 2 pad 4 offset: IP+ 7,0; IP- -7,0 | drill 0.5 pad 0.9: IP+@2 8.89,-0.635; IP+@3 8.89,0.635; IP+@4 8.175,1.625; IP+@5 7,2; IP+@6 5.675,2; IP+@7 4.325,2; IP+@8 3,2; IP+@9 1.825,1.625; IP+@10 1.1,0.625; IP+@11 1.1,-0.625; IP+@12 1.825,-1.625; IP+@13 3,-2; IP+@14 4.325,-2; IP+@15 5.675,-2; IP+@16 7,-2; IP+@17 8.175,-1.625; IP-@2 -8.89,-0.635; IP-@3 -8.89,0.635; IP-@4 -8.175,1.625; IP-@5 -7,2; IP-@6 -5.675,2; IP-@7 -4.325,2; IP-@8 -3,2; IP-@9 -1.825,1.625; IP-@10 -1.1,0.625; IP-@11 -1.1,-0.625; IP-@12 -1.825,-1.625; IP-@13 -3,-2; IP-@14 -4.35,-2; IP-@15 -5.675,-2; IP-@16 -7,-2; IP-@17 -8.175,-1.625
SOIC127P600X175-8N = smd 1.528 x 0.65: 1 -2.711,1.905; 2 -2.711,0.635; 3 -2.711,-0.635; 4 -2.711,-1.905; 5 2.711,-1.905; 6 2.711,-0.635; 7 2.711,0.635; 8 2.711,1.905
SC70 = smd 0.35 x 0.8: 1 -0.65,-0.85; 2 0,-0.85; 3 0.65,-0.85; 4 0.65,0.85; 5 0,0.85; 6 -0.65,0.85
SMA-EDGE = smd 1.524 x 4.064: GND@0 0,0; GND@1 5.08,0; SIG 2.54,0 | smd 1.524 x 4.064 bottom: GND@2 0,0; GND@3 5.08,0
CHIPLED_1206 = smd 1.5 x 1.5: A 0,-1.496; C 0,1.496
SOIC8_150MIL = smd 0.6 x 2.2: 1 -1.905,-2.6; 2 -0.635,-2.6; 3 0.635,-2.6; 4 1.905,-2.6; 5 1.905,2.6; 6 0.635,2.6; 7 -0.635,2.6; 8 -1.905,2.6
5,3//11-PAD = drill 5.3 pad 11: B5,5 0,0
47219-2001_MICROSD = smd 1.45 x 2: P$1 0,0; P$2 13.75,0; P$3 0,8.3; P$4 13.75,8.3 | smd 0.8 x 1.5: PIN1 10.08,2.6; PIN2 8.98,2.6; PIN3 7.88,2.6; PIN4 6.78,2.6; PIN5 5.68,2.6; PIN6 4.58,2.6; PIN7 3.48,2.6; PIN8 2.38,2.6
2/10,16 = drill 2 pad 4: P$1 -5.08,0; P$2 -5.08,10.16; P$3 5.08,0; P$4 5.08,10.16
SOT23-R = smd 0.635 x 1.016: 1 -0.95,-1; 2 0.95,-1; 3 0,1
0207/2V = drill 0.813 pad 1.93: 1 -1.27,0; 2 1.27,0
R0603 = smd 1 x 1.1: 1 -0.85,0; 2 0.85,0
RS-2,5 = drill 0.813 long: 1 -1.27,0; 2 1.27,0
1X03 = drill 1.016 pad 1.88: 1 0,0; 2 2.54,0; 3 5.08,0
SOT223 = smd 1.499 x 2.007: 1 -2.261,-3.15; 2 0.025,-3.15; 3 2.311,-3.15 | smd 3.81 x 2.007: 4 0,3.15
B3F-10XX = drill 1.016 long: 1 -3.251,2.261; 2 3.251,2.261; 3 -3.251,-2.261; 4 3.251,-2.261
SJ = smd 1.168 x 1.6: 1 -0.762,0; 2 0.762,0
SJ_2 = smd 1.168 x 1.6: 1 -1.524,0; 2 0,0; 3 1.524,0
SJ-SMALL = smd 1.016 x 0.508: 1 -0.762,0; 2 0.762,0
STM32F303CB_LQFP48-7X7MM = smd 1.194 x 0.305: 1 -4.25,2.75; 2 -4.25,2.25; 3 -4.25,1.75; 4 -4.25,1.25; 5 -4.25,0.75; 6 -4.25,0.25; 7 -4.25,-0.25; 8 -4.25,-0.75; 9 -4.25,-1.25; 10 -4.25,-1.75; 11 -4.25,-2.25; 12 -4.25,-2.75; 25 4.25,-2.75; 26 4.25,-2.25; 27 4.25,-1.75; 28 4.25,-1.25; 29 4.25,-0.75; 30 4.25,-0.25; 31 4.25,0.25; 32 4.25,0.75; 33 4.25,1.25; 34 4.25,1.75; 35 4.25,2.25; 36 4.25,2.75 | smd 0.305 x 1.194: 13 -2.75,-4.25; 14 -2.25,-4.25; 15 -1.75,-4.25; 16 -1.25,-4.25; 17 -0.75,-4.25; 18 -0.25,-4.25; 19 0.25,-4.25; 20 0.75,-4.25; 21 1.25,-4.25; 22 1.75,-4.25; 23 2.25,-4.25; 24 2.75,-4.25; 37 2.75,4.25; 38 2.25,4.25; 39 1.75,4.25; 40 1.25,4.25; 41 0.75,4.25; 42 0.25,4.25; 43 -0.25,4.25; 44 -0.75,4.25; 45 -1.25,4.25; 46 -1.75,4.25; 47 -2.25,4.25; 48 -2.75,4.25
MA04-1 = drill 1.016 long: 1 -3.81,0; 2 -1.27,0; 3 1.27,0; 4 3.81,0
P1-13 = drill 1.321 pad 2.159 octagon: TP 0,0
P1-13Y = drill 1.321 pad 1.905 long: TP 0,0
TP0.8 = drill 0.8: P$1 0,0
TP0.8_X2 = drill 0.8 long: P$1 0,0; P$2 0,2.54
2/5.08 = drill 1.3 long: P$1 -2.54,0; P$3 2.54,0
RFM12 = smd 1.5 x 3: 1 -5,-10; 2 -3,-10; 3 -1,-10; 4 1,-10; 5 3,-10; 6 5,-10; 7 7,-10; 8 7,6; 9 5,6; 10 3,6; 11 1,6; 12 -1,6; 13 -3,6; 14 -5,6
TP3.5 = drill 3.5 pad 6.096: P$1 0,0
MA06-1 = drill 1.016 long: 1 0,0; 2 2.54,0; 3 5.08,0; 4 7.62,0; 5 10.16,0; 6 12.7,0
CRYSTAL_8X3.8 = smd 1.3 x 1.9: P$1 -2.75,-1.6; P$2 2.75,-1.6; P$3 2.75,1.6; P$4 -2.75,1.6

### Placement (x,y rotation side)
3V3  99.85,40.95 270 top
5V  89.6,41.05 270 top
6V5  88.54,54.32 270 top
BOOT  65.03,17.71 180 top
BOOT1  72.14,38.97 270 top
C1  54.24,56.98 90 top
C2  65.3,62.11 270 top
C3  54.25,44.86 270 top
C4  54.05,31.81 90 top
C5  94.87,24.51 90 top
C6  54.15,19.31 270 top
C7  56.39,56.99 90 top
C8  56.24,31.64 90 top
C9  71.31,43.83 0 top
C10  59.12,30.27 0 top
C11  97.02,24.52 90 top
C12  57.47,16.97 270 top
C13  59.11,55.82 0 top
C14  58.34,43.09 270 top
C15  67.64,30.78 270 top
C16  71.72,41.44 0 top
C17  92.58,24.29 270 top
C18  60.12,50.7 270 top
C19  59.72,25.22 270 top
C20  57.17,61.9 270 top
C21  57.25,67.33 90 top
C22  85.72,58.7 90 top
C23  92.3,58.72 90 top
C24  98.92,58.67 90 top
C25  94.39,6.14 90 bottom
C26  63.05,45.26 90 top
C27  57.26,35.09 180 top
C28  106.81,24.38 270 top
C29  104.65,24.38 270 top
CR1220  73.54,52.04 0 bottom
D1  51.95,69.53 180 top
D2  51.18,55.47 90 top
D3  51.18,46.47 270 top
D4  51.18,29.97 90 top
D5  51.18,20.97 270 top
D7  85.79,45.96 90 top
EBW_A  32.44,25.47 90 top
EBW_B  32.44,50.97 90 top
ESP-12  89.5,24.89 180 top
F1  49.84,73.2 0 top
F2  44.2,56.05 0 top
F3  44.2,45.89 0 top
F4  44.2,30.65 0 top
F5  44.2,20.49 0 top
IC1  25.4,50.97 90 top
IC2  25.4,25.47 90 top
IC3  55.88,25.4 90 top
IC4  56.13,50.93 90 top
INA21X_1  54.22,50.7 90 top
J$1  114.05,25.78 90 top
LED1  109.75,48.65 0 top
LM258  61.77,65.93 180 top
LOGO1  88.31,1.54 0 bottom
MH1  6.35,44.72 0 top
MH2  6.35,57.22 0 top
MH3  6.35,19.22 0 top
MH4  6.35,31.72 0 top
MICRO_SD  67.15,58.69 0 top
MOUNT_10.16_A  11.81,48.39 270 top
MOUNT_10.16_B  11.81,28.07 270 top
Q1  71.6,53.62 180 top
R1  30.97,72.63 0 top
R2  43.94,66.4 270 top
R3  25.05,72.7 0 top
R4  47.01,62.51 90 top
R5  106.16,43.73 180 top
R6  57.79,45.68 0 top
R7  57.46,19.94 0 top
R8  67.94,17.53 0 top
R11  67.74,20.88 180 top
R14  67.73,10.93 0 top
R15  67.75,8.82 180 top
R16  93.51,8.39 90 top
R17  93.94,12.29 0 top
R20  67.73,15.13 0 top
R21  67.73,13.05 0 top
R23  71.89,50.79 0 top
R40  94.23,2.67 180 top
R41  99.31,2.67 180 top
REF_SEL_A  75.68,45.29 0 top
REF_SEL_B  75.71,40.05 0 top
REG1_5V  90.85,47.76 180 top
REG2_3.3  99.85,47.75 180 top
RESET  109.54,16.66 90 top
SJ1  40.96,61.08 0 top
SJ2  51.89,53.04 180 bottom
SJ3  40.98,40.09 180 top
SJ4  37.59,68.33 0 top
SJ5  52.4,28.66 180 bottom
SJ6  72.19,45.96 90 bottom
SJ7  40.95,15.02 0 top
SJ8  47.19,66.32 0 top
SJ9  50.38,63.9 0 top
SJ10  50.15,23.68 270 bottom
SJ11  49.73,49.05 270 bottom
SJ12  95.85,16.92 0 top
SJ13  109.79,44.22 90 top
SJ14  40.98,36.39 0 top
SJ15  14.44,73.09 0 top
SJ16  70.94,45.95 90 bottom
SJ17  69.72,45.97 90 bottom
SJ18  68.45,45.97 90 bottom
SJ19  65.28,33.27 270 bottom
SJ20  64.01,33.27 270 bottom
SJ21  68.33,18.92 0 top
SJ22  69.47,23.62 90 top
SJ23  61.98,8.64 270 bottom
SJ24  63.88,8.64 270 bottom
SJ25  92.33,20.83 0 top
SJ26  92.33,18.92 0 top
SJ27  92.33,16.89 0 top
STM32  64.52,37.97 270 top
SV1  65.76,3.87 0 top
SV2  65.76,1.33 0 top
TP1  59.35,59.31 0 top
TP8  17.53,21.84 90 top
TP9  17.53,29.46 90 top
TP10  17.53,47.24 90 top
TP11  17.53,54.86 270 top
U$1  49.64,66.25 0 top
U$2  63.37,71.78 0 top
U$3  104.01,56.54 0 top
U$4  52.75,63.87 0 top
U$5  59.5,27.89 0 top
U$6  60.11,53.45 0 top
U$7  87.84,44.53 0 top
U$8  102.85,44.67 0 top
U$9  86.65,51.16 0 top
U$10  104.01,71.78 0 top
U$11  63.37,56.54 0 top
U$12  88.83,69.28 180 top
U$13  26.93,8.46 0 top
U$14  103.63,35.31 270 top
U$18  93.76,44.47 0 top
U$19  96.81,44.48 0 top
U$21  27.73,67.61 0 top
U$22  17.36,9.36 0 top
U$23  99.36,9.36 0 top
U$24  17.36,67.36 0 top
U$25  99.36,67.36 0 top
U$26  38.44,7.02 270 top
UART/ESP  87.25,28.25 180 top
UART/STM  87.26,32.06 180 top
Y1  65.9,50.75 90 top

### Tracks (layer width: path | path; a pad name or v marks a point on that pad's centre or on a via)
3.3V_PRE
  Top 0.406: C24.1 99.83,55.79 99.83,51.13 | 99.83,51.13 REG2_3.3.2 | 99.91,40.12 99.85,40.17 3V3.1 REG2_3.3.4 | REG2_3.3.4 96.93,44.6 U$19.P$1 | REG2_3.3.4 99.92,44.67 U$8.P$1 | REG2_3.3.4 99.85,51.1 99.83,51.13
5V_PRE
  Top 0.406: U$12.P$1 91.37,64.67 89.69,62.99 89.69,59.34 C23.1 92.3,56.09 90.83,54.62 REG1_5V.2 90.83,44.64 REG1_5V.4 | 90.99,44.47 REG1_5V.4 | 91.14,44.53 91.17,44.5 | 91.17,44.5 91.2,44.47 | D7.C U$7.P$1 87.91,44.61 REG1_5V.4 | 89.71,41.92 5V.1 89.6,43.08 90.99,44.47 | U$18.P$1 90.99,44.47 | 91.17,44.5 91.15,44.48 REG1_5V.4
6.5V
  Top 0.406: C22.1 85.72,55.1 87.27,53.54 88.52,53.54 6V5.2 REG1_5V.3 88.39,51.13 86.72,51.13 U$9.P$1
+3V3  (via drill 0.5)
  Top 0.203: INA21X_1.3 55.46,51.73 v55.85,51.73
  Top 0.254: C27.1 58.16,35.04 59.24,35.04 v59.24,34.71 59.24,35.12 59.34,35.22 STM32.24 | STM32.36 v67.27,32.64 67.27,32.01 C15.1 | STM32.48 v69.89,40.72 70.16,40.72 C16.1 | STM32.9 63.27,44.2 C26.1 63.71,44.41 v64.03,44.73 | R20.1 v66.88,14.06 R21.1 | 93.57,10.36 93.57,11.05 94.79,12.27 R17.2 | 93.57,10.36 93.57,9.3 R16.2 | v93.5,10.36 93.57,10.36 | 102.79,40.19 102.81,40.18 v103.02,39.78
  Top 0.406: MICRO_SD.PIN4 73.93,59.93 v73.99,59.88 | R23.2 72.72,50.77 v72.72,49.69 | 90.42,22.89 ESP-12.16 89.57,22.96 v89.57,24.13 | 90.42,22.89 92.03,22.89 C17.2 94.69,23.44 | 94.69,23.44 94.74,23.44 C5.1 C11.1 97.02,23.47 v95.97,22.42 | 3V3.2 102.43,40.19 | 102.43,40.19 102.96,40.72 102.96,41.38 | 102.96,41.38 R5.2 | C16.1 70.87,42.19 v70.66,42.52 70.59,43.6 C9.1 | v102.96,41.4 102.96,41.38 | v103.02,39.78 102.61,40.19 102.43,40.19 | v98.23,40.61 98.65,40.19 99.24,40.19 98.64,39.59 v98.31,39.59 | v94.87,22.31 95.7,22.31 95.76,22.37 94.69,23.44 | v91.23,23.71 90.42,22.89 | C29.1 105.41,25.33 | 105.41,25.33 C28.1 | C28.1 106.68,25.46 106.68,27.94 | 106.68,27.94 v106.68,30.48 109.46,30.48 U$14.9 | C28.1 105.78,26.36 v105.78,26.54 | 105.41,25.33 v105.41,27.94 106.68,27.94
  +3V3 0.406: v105.78,26.54 104.64,25.4 104.14,25.4
  Bottom 0.254: v93.5,10.36 93.5,3.2 R40.2
  Bottom 0.406: SJ11.3 49.73,46.74 v49.01,46.02 | SJ10.3 48.87,20.88 v48.87,20.03
  pour +3V3 (isolate 0.356): 48.76,87.63 126.25,87.63 126.25,-7.62 48.76,-7.62
+3V3_BAT
  Top 0.406: R23.1 71.04,52.06 Q1.3
+5V  (via drill 0.5)
  Top 0.406: UART/ESP.4 UART/STM.4 79.64,32.28 83.42,36.07 83.5,36.2 85.09,36.2 89.06,40.16 89.48,40.16 5V.2 90.2,40.29 91.69,41.78 92.58,41.78 93.98,43.18 95.25,43.18 95.25,46.88 94.34,47.8 | v89.49,47.84 88.27,47.84 79.14,56.98 79.14,62.64 78.04,63.73 66.07,63.73 C2.1 64.04,62.96 LM258.8 | C10.1 57.97,30.27 v57.15,29.45 56.52,28.82 IC3.6 | C13.1 57.41,54.97 v57.41,54.92 56.77,54.28 IC4.6 56.83,53.5 v56.83,52.23 | 94.34,47.8 v92.09,47.8 | 94.34,47.8 94.43,47.8 REG2_3.3.3
  Bottom 0.406: v92.09,47.8 89.53,47.8 v89.49,47.84 | 58.55,30.92 61.25,28.22 61.25,27.11 60.5,26.36 | 58.55,30.92 54.41,35.06 54.41,46.41 50.29,50.52 49.76,50.52 SJ11.1 50.32,50.64 51.44,50.64 51.59,50.8 53.18,50.8 54.93,52.55 56.52,52.55 v56.83,52.23 | 60.5,26.36 59.36,25.22 50.22,25.22 SJ10.1 | 60.5,26.36 60.66,26.29 77.72,26.29 79.63,28.19 UART/ESP.4 | v57.15,29.45 57.15,29.53 58.42,30.8 58.55,30.92
ADC
  Top 0.203: ESP-12.10 89.72,10.89 91.5,9.11 91.5,6.73 95.5,2.72 R40.1 R41.2
  Bottom 0.203: C25.1 94.49,5.24 94.49,3.62 95.44,2.67 R40.1
ADCSHUNT_OUT_A  (via drill 0.5)
  Top 0.203: STM32.10 62.77,42.29 62.77,43.15 60.96,44.96 60.96,50.77 60.2,51.53 C18.1 60.1,51.63 60.1,53.44 U$6.P$1 60.01,53.44 59.82,53.63 58.1,53.63 IC4.5 | INA21X_1.6 53.88,50.05 54.25,50.41 54.25,51.97 53.68,52.54 v53.15,52.54
  Bottom 0.203: 52.67,53.05 59.72,53.05 60.1,53.44 U$6.P$1 | 52.67,53.05 SJ2.2 | v53.15,52.54 52.67,53.01 52.67,53.05
ADCSHUNT_OUT_B  (via drill 0.5)
  Top 0.203: C19.1 59.63,26.1 59.63,27.72 59.53,27.81 U$5.P$1 | v61.72,36.48 61.72,42.2 STM32.12 | v61.34,29.24 59.72,27.62 U$5.P$1 | IC3.5 57.82,28.1 59.24,28.1 59.44,27.91 U$5.P$1
  Bottom 0.203: v61.72,36.48 61.72,30.67 61.82,30.57 61.82,29.72 v61.34,29.24 | SJ5.2 53.24,28.57 58.77,28.57 59.44,27.91 U$5.P$1
ANT
  Top 0.813: J$1.SIG 114.03,28.31 U$14.8
BOOT_STM
  Top 0.254: STM32.44 70.81,38.72 BOOT1.1
CH_PD
  Top 0.203: R17.1 93,12.55 89.85,12.55 89.53,12.86 ESP-12.11
D0/RX
  Top 0.203: ESP-12.8 74.56,8.89 84.68,19 84.68,28.19 UART/ESP.2
D1/TX
  Top 0.203: ESP-12.7 73.27,10.93 R14.2 68.58,8.83 R15.1
GND  (via drill 0.5)
  Top 0.203: INA21X_1.2 56.08,50.7 v56.15,50.76
  Top 0.254: STM32.8 63.77,43.16 v64.16,43.55 | STM32.47 66.52,40.22 64.48,38.18 | STM32.35 66.77,35.9 64.48,38.18 | STM32.23 62.02,35.72 v64.4,38.1 64.48,38.18
  other vias: 65.84,7.69 55.27,21.36 52.99,17.98 49.28,18.03 49.66,16.91 55.1,32.65 55.22,35.73 52.82,33.66 49.81,33.87 49.33,33.05 49.24,43.42 49.8,42.45 52.62,42.67 53.03,43.83 49.37,58.47 49.67,59.53 52.63,59.4 55.34,58.02 60.75,55.29 55.54,46.82 67.58,28.94 65.82,21.54 74.87,22.89 75.82,22.91 71.72,22.89 73.27,24.16 93.62,25.42 95.48,26.82 97.03,26.79 107.98,50.36 102.18,52.51 103.29,52.33 92.46,52.62 93.7,52.53 86.67,59.59 93.43,59.68 100.07,59.42 98.01,59.67 91.32,59.74 84.69,59.6 79.67,68.42 67.91,68.66 65.88,58.76 58.72,68.45 56.14,61.15 47.93,70.16 47.85,69.32 43.09,40.84 43.17,40 43.07,38.98 43.07,38.01 43.22,37 43.25,36.16 43.4,15.67 43.33,14.57 43.01,13.35 42.86,59.73 43.1,60.75 43.07,61.83 86.17,48.71 85.07,48.73 72.56,42.52 72.58,55.77 57.65,41.15 57.58,14.91 91.18,25.59 92.31,26.14 22.64,8.69 22.41,7.33 23.11,5.55 24.74,5.64 28.49,5.49 30.39,5.55 31.11,11.02 27.77,8.9 27.68,7.21 84.79,71.54 84.43,70.43 84.38,69.22 84.49,67.84 85.21,66.76 104.05,60.67 105.36,60.48 106.23,59.2 105.96,58.02 106.23,56.41 105.6,55.13 64.23,57.84 63.35,57.83 62.47,57.86 71.69,62.59 80.9,60.64 33.84,68 78.4,36.27 61.14,30.26 107.07,32.63 107.19,31.61 112.02,32.63 113.04,32.5 114.05,32.63 115.45,32.5 111,26.28 111,25.26 111.51,24.37 113.04,23.99 114.69,23.99 115.83,23.99 96.04,28.96 91.36,28.34 96.73,29.69 91.35,29.41
  pour Bottom (isolate 0.254, rank 3): -5.59,80.53 -5.59,64.11 41.97,64.11 41.97,11.96 -4.8,11.96 -4.8,-7.37 125.18,-7.37 128.78,80.53
  pour Top (isolate 0.203, rank 3): -3.52,78.74 -3.52,64.24 41.57,64.24 41.57,12.46 -4.27,12.46 -4.27,-3.56 105.02,-3.56 123.54,16.82 123.54,63.44 109.64,78.74
  pour GND (isolate 0.356, rank 3): -0.69,78.74 -0.69,64.24 41.57,64.24 41.57,12.46 -1.63,12.46 -1.63,-3.56 105.02,-3.56 122.34,15.5 122.34,64.77 109.64,78.74
GPIO0
  Top 0.203: ESP-12.4 73.25,16.86 70.2,16.86 69.63,16.29 63.91,16.29 62.58,17.62 BOOT.2
GPIO2
  Top 0.203: R8.2 68.87,17.53 69.06,17.72 69.06,18.86 SJ21.2 69.15,18.95 73.25,18.95 ESP-12.3
GPIO2_STM
  Top 0.203: SJ21.1 67.63,18.95 67.63,20.1 67.72,20.19 67.72,24.57 68.67,25.53 68.67,35.15 STM32.37
GPIO12  (via drill 0.5)
  Top 0.203: v71.06,59.91 71.06,60.39 70.67,60.77 70.67,61.25 MICRO_SD.PIN7 | SJ26.2 93.66,18.92 v94.13,19.39 | v88.9,37.47 91.44,40.01 93.34,40.01 U$14.1
  Bottom 0.203: 69.72,47.91 69.72,50.77 71.06,52.1 v71.06,59.91 | 69.72,47.91 SJ17.2 | v94.13,19.39 94.13,19.54 90.3,23.38 90.3,32.96 88.93,34.32 | 88.93,34.32 79.25,44.01 77.72,44.01 76.96,44.77 76.96,45.81 74.87,47.91 69.72,47.91 | v88.9,37.47 88.9,34.29 88.93,34.32
GPIO12_ESP
  Top 0.203: SJ26.1 91.53,18.95 89.53,18.95 ESP-12.14
GPIO13  (via drill 0.5)
  Top 0.203: v93.23,21.7 93.23,20.96 SJ25.2 93.34,20.95 97.16,20.95 99.06,22.86 99.06,27.94 107.31,36.2 109.22,36.2 U$14.12 | MICRO_SD.PIN3 75.06,61.25 v75.06,52.77 73.15,52.77 71.91,51.53 71.91,50.1 71.25,49.44 v69.06,49.44
  Bottom 0.203: v93.23,21.7 93.23,24.88 92.96,25.15 92.96,25.81 93.06,25.91 93.06,34.77 v75.06,52.77 | v69.06,49.44 68.48,48.86 68.48,46.77 SJ18.2
GPIO13_ESP
  Top 0.203: SJ25.1 91.53,20.86 89.53,20.86 ESP-12.15
GPIO14  (via drill 0.5)
  Top 0.203: v93.03,17.72 93.06,16.95 SJ27.2 | v76.96,43.72 76.96,45.81 77.92,46.77 77.92,62.2 77.72,62.39 73.44,62.39 72.87,61.82 72.87,61.34 MICRO_SD.PIN5 | v97.79,38.1 109.22,38.1 U$14.13 | v90.81,38.1 90.76,38.1 87.47,34.81 v86.76,34.81
  Bottom 0.203: v93.03,17.72 92.84,17.91 92.84,18.33 88.39,22.78 88.39,34.29 87.31,35.37 | 87.31,35.37 79.06,43.62 76.96,43.62 | 76.96,43.62 75.53,43.62 73.72,45.43 73.72,46.39 72.58,47.53 71.72,47.53 70.96,46.77 SJ16.2 | v76.96,43.72 76.96,43.62 | v90.81,38.1 v97.79,38.1 | 87.31,35.37 v86.76,34.81
GPIO14_ESP
  Top 0.203: SJ27.1 91.53,16.86 89.53,16.86 ESP-12.13
GPIO15  (via drill 0.5)
  Top 0.203: 74.39,46.1 74.39,51.15 76.11,52.86 76.11,61.25 MICRO_SD.PIN2 | 74.39,46.1 74.39,39.62 74.77,39.24 74.77,35.72 69.53,30.48 69.53,24.38 SJ22.2 | 74.39,46.1 v73.06,46.1
  Bottom 0.203: v73.06,46.1 72.48,46.67 72.2,46.67 SJ6.2
GPIO15_ESP
  Top 0.203: 69.44,21.72 69.44,22.86 SJ22.1 | 69.44,21.72 68.67,20.95 R11.1 | ESP-12.2 73.25,20.95 70.29,20.95 69.53,21.72 69.44,21.72
GPIO16
  Top 0.203: SJ12.1 95.09,16.35 93.69,14.95 89.53,14.95 ESP-12.12
I2C1_SCL  (via drill 0.5)
  Top 0.203: v67.53,36.29 67.53,37.15 68.1,37.72 68.67,37.72 STM32.42
  Bottom 0.203: v67.53,36.29 SJ19.1
I2C1_SDA  (via drill 0.5)
  Top 0.203: v66.86,36.96 67.15,37.24 67.15,37.34 68.01,38.2 68.67,38.2 STM32.43
  Bottom 0.203: v66.86,36.96 64.01,34.1 SJ20.1
LOAD_A  (via drill 0.5)
  Top 0.406: 39.62,40.08 40.16,40.08 SJ3.2 | v36.2,65 37.49,65 39.17,66.67 39.17,68.28 SJ4.3
  Bottom 0.406: 37.16,45.87 41.6,45.87 F3.1 | v36.2,65 36.2,64.47 38.25,62.41 38.25,51.21 37.19,50.14 37.16,50.14
  pour Top (no thermals): 0.35,50.22 39.62,50.22 39.62,39.22 0.35,39.22
  pour Bottom (isolate 0.813, no thermals): 37.16,50.22 0.35,50.22 0.35,39.22 37.16,39.22
LOAD_B  (via drill 0.5)
  Top 0.406: v36.96,66.37 36.73,66.37 36.04,67.06 36.04,68.28 SJ4.1 | 39.61,20.5 41.6,20.5 F5.1
  Bottom 0.406: v36.96,66.37 36.96,66.14 39.78,63.32 39.78,51.36 43.51,47.62 43.51,43.2 38.25,37.95 38.25,25.76 37.19,24.69 37.16,24.69
  pour Top (no thermals): 0.35,24.72 39.61,24.72 39.61,14.17 0.35,14.17
  pour Bottom (isolate 0.813, no thermals): 37.16,24.72 0.35,24.72 0.35,14.23 37.16,14.23
LOAD_B_T
  Top 0.254: IC3.1 53.8,22.78 51.59,22.78 51.21,23.16 D5.C 51.05,23.16 49.45,23.16 46.79,20.5 F5.2
  Top 0.406: C6.1 53.98,20.34 IC3.1
LOAD_T_A
  Top 0.203: INA21X_1.5 51.84,50.7 51.21,50.06 51.21,48.62
  Top 0.254: C3.1 54.25,48.16 IC4.1 54.1,48.23 51.59,48.23 51.21,48.62 D3.C 51.05,48.69 50.67,48.69 47.93,45.95 46.79,45.95 F3.2
N$1
  Top 0.203: F1.P$2 44.77,73.25 39.72,73.25 F1.P$1
  Top 0.406: SJ15.2 14.44,74.68 15.57,75.81 36.98,75.81 F1.P$1 37.59,71.21 SJ4.2
N$3
  Top 0.203: IC4.4 58.04,46.27 R6.2 58.34,45.38 C14.1
N$4
  Top 0.203: C18.2 60,49.73 57.52,49.73 56.77,48.97 IC4.3 56.94,48.05 R6.1
N$5
  Top 0.203: R5.1 107.27,43.48 109.77,43.48 SJ13.1
N$6
  Top 0.203: LED1.A 109.82,47.12 109.82,45.41 SJ13.2
N$25
  Top 0.203: R7.1 56.6,22.6 IC3.3 56.63,22.8 56.63,24.11 56.9,24.37 C19.2
N$27
  Top 0.203: C12.1 58.3,18.65 R7.2 58.3,22.17 IC3.4
N$29  (via drill 0.5)
  Top 0.203: v69.72,15.24 68.67,15.24 68.58,15.14 R20.2
  Bottom 0.203: v69.72,15.24 67.06,15.24 62.01,10.19 62.01,9.43 SJ23.1
N$30  (via drill 0.5)
  Top 0.203: v65.82,11.05 65.82,11.34 66.67,12.19 67.63,12.19 68.48,13.05 R21.2
  Bottom 0.203: v65.82,11.05 64.2,9.43 63.91,9.43 SJ24.1
N$36
  Top 0.203: R14.1 66.96,10.95 67.15,10.95 68.39,12.19 70.01,12.19 71.71,13.9 74.56,13.9 82.11,21.45 82.11,28.19 UART/ESP.3
N$37  (via drill 0.5)
  Top 0.203: INA21X_1.1 55.74,50.05 v56.11,49.67
  Bottom 0.203: v56.11,49.67 58.66,52.22 60.63,52.22 61.05,52.65 61.05,54.04 59.3,55.78 59.3,59.27 TP1.TP
OSC32_IN
  Top 0.203: STM32.3 66.27,46.77 Y1.P$1
OSC32_OUT
  Top 0.203: STM32.4 65.77,46.53 Y1.P$4
REF_A_INPUT  (via drill 0.5)
  Top 0.203: IC4.7 55.53,53.72 55.53,54.01 56.39,54.86 56.39,56.1 C7.1 56.48,56.2 57.05,56.2 57.63,56.77 61.25,56.77 62.58,55.44 71.06,55.44 71.72,54.77 v71.72,53.72
  Bottom 0.203: v71.72,53.72 71.72,51.82 78.2,45.34 REF_SEL_A.2
REF_B_INPUT
  Top 0.203: IC3.7 55.24,28.38 56.2,29.34 56.2,30.77 C8.1 56.29,30.86 57.34,30.86 57.63,31.15 61.25,31.15 65.15,27.24 65.15,20.1 66.86,18.38 67.72,18.38 68.01,18.1 68.01,16.86 68.2,16.67 69.44,16.67 70.77,18 74.49,18 78.2,21.72 78.2,35.53 77.72,36.01 77.72,39.53 78.2,40.01 REF_SEL_B.2
RFM_IRQ  (via drill 0.5)
  Top 0.203: STM32.2 66.77,43.33 v67.35,43.92 | v83.43,34.31 85.95,34.31 86.29,33.97 88.58,33.97 91.51,36.9 91.51,37.29 92.35,38.13 93.46,38.13 U$14.2
  Bottom 0.203: v67.35,43.92 64.15,40.72 64.15,39.89 65.51,38.53 66.74,38.53 70.81,34.46 83.27,34.46 v83.43,34.31
RFM_SEL  (via drill 0.5)
  Top 0.203: U$14.14 104.51,40.31 103.11,38.91 98.03,38.91 97.57,39.37 v96.52,39.37 | v87.89,42 86.72,42 80.66,35.94 v80.13,35.94 | v76.06,35.79 75.76,35.79 70.55,30.58 v70.55,30.17 | v65.01,30.47 64.46,30.47 v62.78,32.15 | v64.16,35.64 65.3,35.64 66.28,34.65 66.28,33.74 STM32.34
  Bottom 0.203: v96.52,39.37 90.52,39.37 v87.89,42 | v80.13,35.94 79,35.94 78.67,35.62 76.23,35.62 v76.06,35.79 | v70.55,30.17 65.31,30.17 v65.01,30.47 | v62.78,32.15 62.78,34.26 v64.16,35.64
RST  (via drill 0.5)
  Top 0.203: 96.58,13.43 96.58,11.34 94.39,9.14 94.39,8.48 93.53,7.62 R16.1 93.53,7.71 92.58,8.67 92.58,10.11 90.77,11.93 88.18,11.93 88.07,11.82 | 96.58,13.43 96.58,16.86 SJ12.2 | 88.07,11.82 87.93,11.68 87.93,9.95 89.04,8.89 ESP-12.9 | 96.58,13.43 107.25,13.43 RESET.1 | v65.53,40.29 64.29,41.53 64.29,42.2 STM32.7 | UART/STM.1 87.34,32 87.34,28.29 UART/ESP.1 87.34,28.19 87.34,12.54 88.07,11.82
  Bottom 0.203: v65.53,40.29 66.01,40.29 71.22,35.08 85.27,35.08 86.86,33.48 UART/STM.1
SCL  (via drill 0.5)
  Top 0.203: ESP-12.6 73.23,12.81 v71.68,12.81 | SV2.2 64.58,1.43 64.58,3.81 SV1.2
  Bottom 0.203: SV1.2 64.48,3.9 63.91,4.48 63.91,7.81 SJ24.2 64.13,7.38 70.56,13.81 | 70.56,13.81 80.77,24.02 80.77,29.15 81.15,29.53 81.15,30.48 81.06,30.57 81.06,32.96 80.11,33.91 67.53,33.91 66.2,32.58 65.34,32.58 SJ19.2 | 70.56,13.81 71.56,12.81 v71.68,12.81
SDA  (via drill 0.5)
  Top 0.203: v64.01,27.15 64.01,21.05 61.25,18.29 61.25,4.57 61.91,3.9 SV1.1 62.01,3.81 62.01,1.43 SV2.1 | v69.53,14.1 70.29,14.86 73.25,14.86 ESP-12.5
  Bottom 0.203: SV1.1 62.01,3.9 62.01,7.81 SJ23.2 62.91,8.81 62.91,9.93 63.75,10.77 64.58,10.77 67.91,14.1 v69.53,14.1 | v64.01,27.15 SJ20.2
SOURCE_A
  Top 0.406: 39.59,61.11 40.16,61.11 SJ1.1 | 39.59,56.08 41.6,56.08 F2.1
  pour Bottom (isolate 0.813, no thermals): 37.16,61.93 0.35,61.93 0.35,51.72 37.16,51.72
  pour Top (no thermals): 0.35,62.02 39.59,62.02 39.59,51.72 0.35,51.72
SOURCE_B
  Top 0.406: 39.63,36.42 40.16,36.42 SJ14.1 | 39.63,30.71 41.6,30.71 F4.1
  pour Bottom (isolate 0.813, no thermals): 37.16,37.22 0.35,37.22 0.35,26.22 37.16,26.22
  pour Top (no thermals): 0.35,37.22 39.63,37.22 39.63,26.22 0.35,26.22
SOURCE_B_T
  Top 0.254: IC3.8 53.8,28.04 51.44,28.04 51.21,27.81 D4.C 51.05,27.81 49.61,27.81 46.79,30.63 F4.2
  Top 0.406: IC3.8 53.98,30.89 C4.1
SOURCE_T_A
  Top 0.203: INA21X_1.4 53.1,51.35 D2.C
  Top 0.254: C1.1 54.25,56.08 54.25,53.65 IC4.8 54.1,53.65 51.51,53.65 51.21,53.34 D2.C 51.13,53.42 48.54,56.01 46.79,56.01 F2.2
SPI_CLK  (via drill 0.5)
  Top 0.203: v73.44,39.81 73.44,35.91 72.68,35.15 70.58,35.15 69.53,36.2 68.77,36.2 STM32.39
  Bottom 0.203: v73.44,39.81 71.82,41.43 71.82,42.39 70.96,43.24 70.96,45.15 SJ16.1
SPI_CSS  (via drill 0.5)
  Top 0.203: v74.11,36.01 72.87,34.77 70.39,34.77 69.44,35.72 STM32.38
  Bottom 0.203: v74.11,36.01 74.11,41.91 72.2,43.81 72.2,45.15 SJ6.1
SPI_MISO  (via drill 0.5)
  Top 0.203: v70.67,37.91 70.67,36.96 70.29,36.58 69.63,36.58 69.53,36.67 68.77,36.67 STM32.40
  Bottom 0.203: SJ17.1 69.72,41.91 70.67,40.96 v70.67,37.91
SPI_MOSI  (via drill 0.5)
  Top 0.203: v70.01,37.24 68.77,37.24 STM32.41
  Bottom 0.203: v70.01,37.24 68.48,38.77 68.48,45.15 SJ18.1
USART1_RX  (via drill 0.5)
  Top 0.203: v66.48,31.34 64.77,33.05 STM32.31 | v80.49,30.19 80.49,30.39 82.11,32 UART/STM.3
  Bottom 0.203: v66.48,31.34 72.96,31.34 74.11,30.19 v80.49,30.19
USART1_TX  (via drill 0.5)
  Top 0.203: v67.63,25.43 65.83,27.23 65.83,30.9 64.29,32.43 64.29,33.72 STM32.30 | v79.15,25.43 81.06,27.34 81.06,29.43 81.82,30.19 82.87,30.19 84.68,32 UART/STM.2
  Bottom 0.203: v79.15,25.43 v67.63,25.43
V+_A  (via drill 0.5)
  Top 0.406: U$21.P$3 30.27,72.06 R1.1 | v12.3,71.5 12.3,72.48 12.89,73.06 | 12.89,73.06 12.89,73.09 | SJ15.1 12.88,73.08 12.89,73.06
  Bottom 0.406: U$21.P$3 30.27,72.02 27.42,74.87 15.67,74.87 v12.3,71.5
V+_B
  Top 0.406: R3.1 23.78,69.02 U$21.P$1 19.71,73.09 SJ15.3
V_IN_POSTFUSE
  Top 0.406: 63.4,73.15 63.4,74.3 U$2.P$2 | 63.4,73.15 63.4,71.86 U$2.P$1 | 63.4,73.15 60.12,73.15 F1.P$3 59.89,73.23 55.09,73.23 F1.P$4 54.86,73.15 54.56,72.85 54.56,69.57 D1.C
VBAT  (via drill 0.5)
  Top 0.203: 69.58,53.58 68.39,52.39 68.39,49.15 68.77,48.77 68.77,43.72 67.34,42.29 STM32.1 | 69.58,53.58 70.58,54.58 Q1.2 | v69.53,53.63 69.58,53.58
  Bottom 0.203: v69.53,53.63 69.53,53.58
  Bottom 0.406: 70.57,53.58 69.53,53.58 66.78,53.58 CR1220.P+
VCC_ACS_A
  Bottom 0.254: IC1.1 49.28,49.06 49.51,48.83 SJ11.2
VCC_ACS_B
  Bottom 0.254: IC2.1 50.03,23.56 SJ10.2
VOUT_ACS_A
  Bottom 0.203: SJ2.1 51.05,52.96 46.86,52.96 IC1.3
VOUT_ACS_B
  Bottom 0.203: SJ5.1 51.63,28.57 48.01,28.57 46.86,27.43 IC2.3
VOUT_POST_SWITCHING
  Top 0.406: U$10.P$1 U$10.P$2 93.38,74.33 93.02,74.68 92.15,74.68 88.16,70.69 88.16,55.47 6V5.1
VSENSE_A
  Top 0.203: SJ8.1 46.39,66.29 45.15,66.29 44.01,65.15 R2.2
  Bottom 0.203: R1.2 32.29,72.58 36.48,72.58 43.91,65.15 R2.2
VSENSE_A_BUFFED  (via drill 0.5)
  Top 0.203: v61.53,43.43 61.72,43.43 62.2,42.96 62.2,42.29 STM32.11 | v61.53,66.86 61.53,67.06 62.39,67.91 62.39,68.48 LM258.2 62.48,68.58 63.63,68.58 LM258.1
  Bottom 0.203: v61.53,66.86 v61.53,43.43
VSENSE_A_TP
  Top 0.203: SJ8.2 48.01,66.29 49.62,66.29 U$1.P$1 49.72,66.29 57.15,66.29 57.24,66.39 C21.1 57.34,66.48 59.63,66.48 61.05,67.91 61.05,68.48 LM258.3
VSENSE_B
  Top 0.203: SJ9.1 49.53,63.82 47.05,63.82 R4.2 46.96,63.72 30.57,63.72 28.38,65.91 28.38,68.01 26.38,70.01 26.38,72.68 R3.2
VSENSE_B_BUFFED
  Top 0.203: STM32.13 60.2,40.67 58.1,40.67 57.91,40.48 49.53,40.48 45.53,44.48 45.53,57.44 50.01,61.91 60.29,61.91 61.05,62.67 61.05,63.25 LM258.6 61.15,63.34 62.39,63.34 LM258.7
VSENSE_B_TP
  Top 0.203: LM258.5 59.82,63.25 59.34,62.77 57.24,62.77 C20.1 57.15,62.77 53.82,62.77 52.77,63.82 U$4.P$1 52.67,63.91 51.15,63.91 SJ9.2

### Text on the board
bPlace: emonDC | wireless energy monitoring node | Technology that helps us live within ecological limits | OpenEnergyMonitor.org | Designed in / North Wales / by Daniel Bates | Open / Hardware
tNames: A | B | 5V_IN | +6.5V_IN | +OUT | GND | GND | 5V | Vsense | Vsense | 1 | Vout | A | PWR_OK | Vcc | BI | UNI | UNI | BI | 2 | TR5 / FUSES | 1 | UART/STM | GND | Vout | 5V | Rx | Tx | RST | B | ESP | Vcc | 2 | STM_v0.1 / DEC 2019 / by DB | 5.08mm | GND | GND | emonDC / _duo_ | SCL | SDA | 3V3 | I2C | Wireless Energy / Monitoring Node | GND | 3.3V | GND | 1V
bNames: 5V | 3V3 | 5V | 3V3
_tsilk: Designed in | North Wales | Made in UK
_bsilk: SMT V0.6 rev3 | emonTx | wireless energy monitoring node | SMT V0.6 rev3 | emonTx | SMT V0.6 rev3 | emonTx | Technology that helps us live within ecological limits | wireless energy monitoring node | wireless energy monitoring node | Designed in North Wales UK by Glyn Hudson & Trystan Lea | Technology that helps us live within ecological limits | Technology that helps us live within ecological limits | Designed in North Wales UK by Glyn Hudson & Trystan Lea | 165mm ant | 433Mhz | Designed in North Wales UK by Glyn Hudson & Trystan Lea | 165mm ant | 165mm ant | 433Mhz | 433Mhz | 868Mhz | 82mm ant | 82mm ant | 82mm ant | 868Mhz | 868Mhz | 78mm ant | 915Mhz | 78mm ant | 915Mhz | 78mm ant | 915Mhz | 165mm ant | 433Mhz | 82mm ant | 868Mhz | 78mm ant | 915Mhz

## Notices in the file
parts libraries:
SparkFun-Connectors: Licensing: CC v3.0 Share-Alike You are welcome to use this library for commercial purposes.
microbuilder: This work is placed in the public domain, and may be freely used for commercial and non-commercial work with the following conditions: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
